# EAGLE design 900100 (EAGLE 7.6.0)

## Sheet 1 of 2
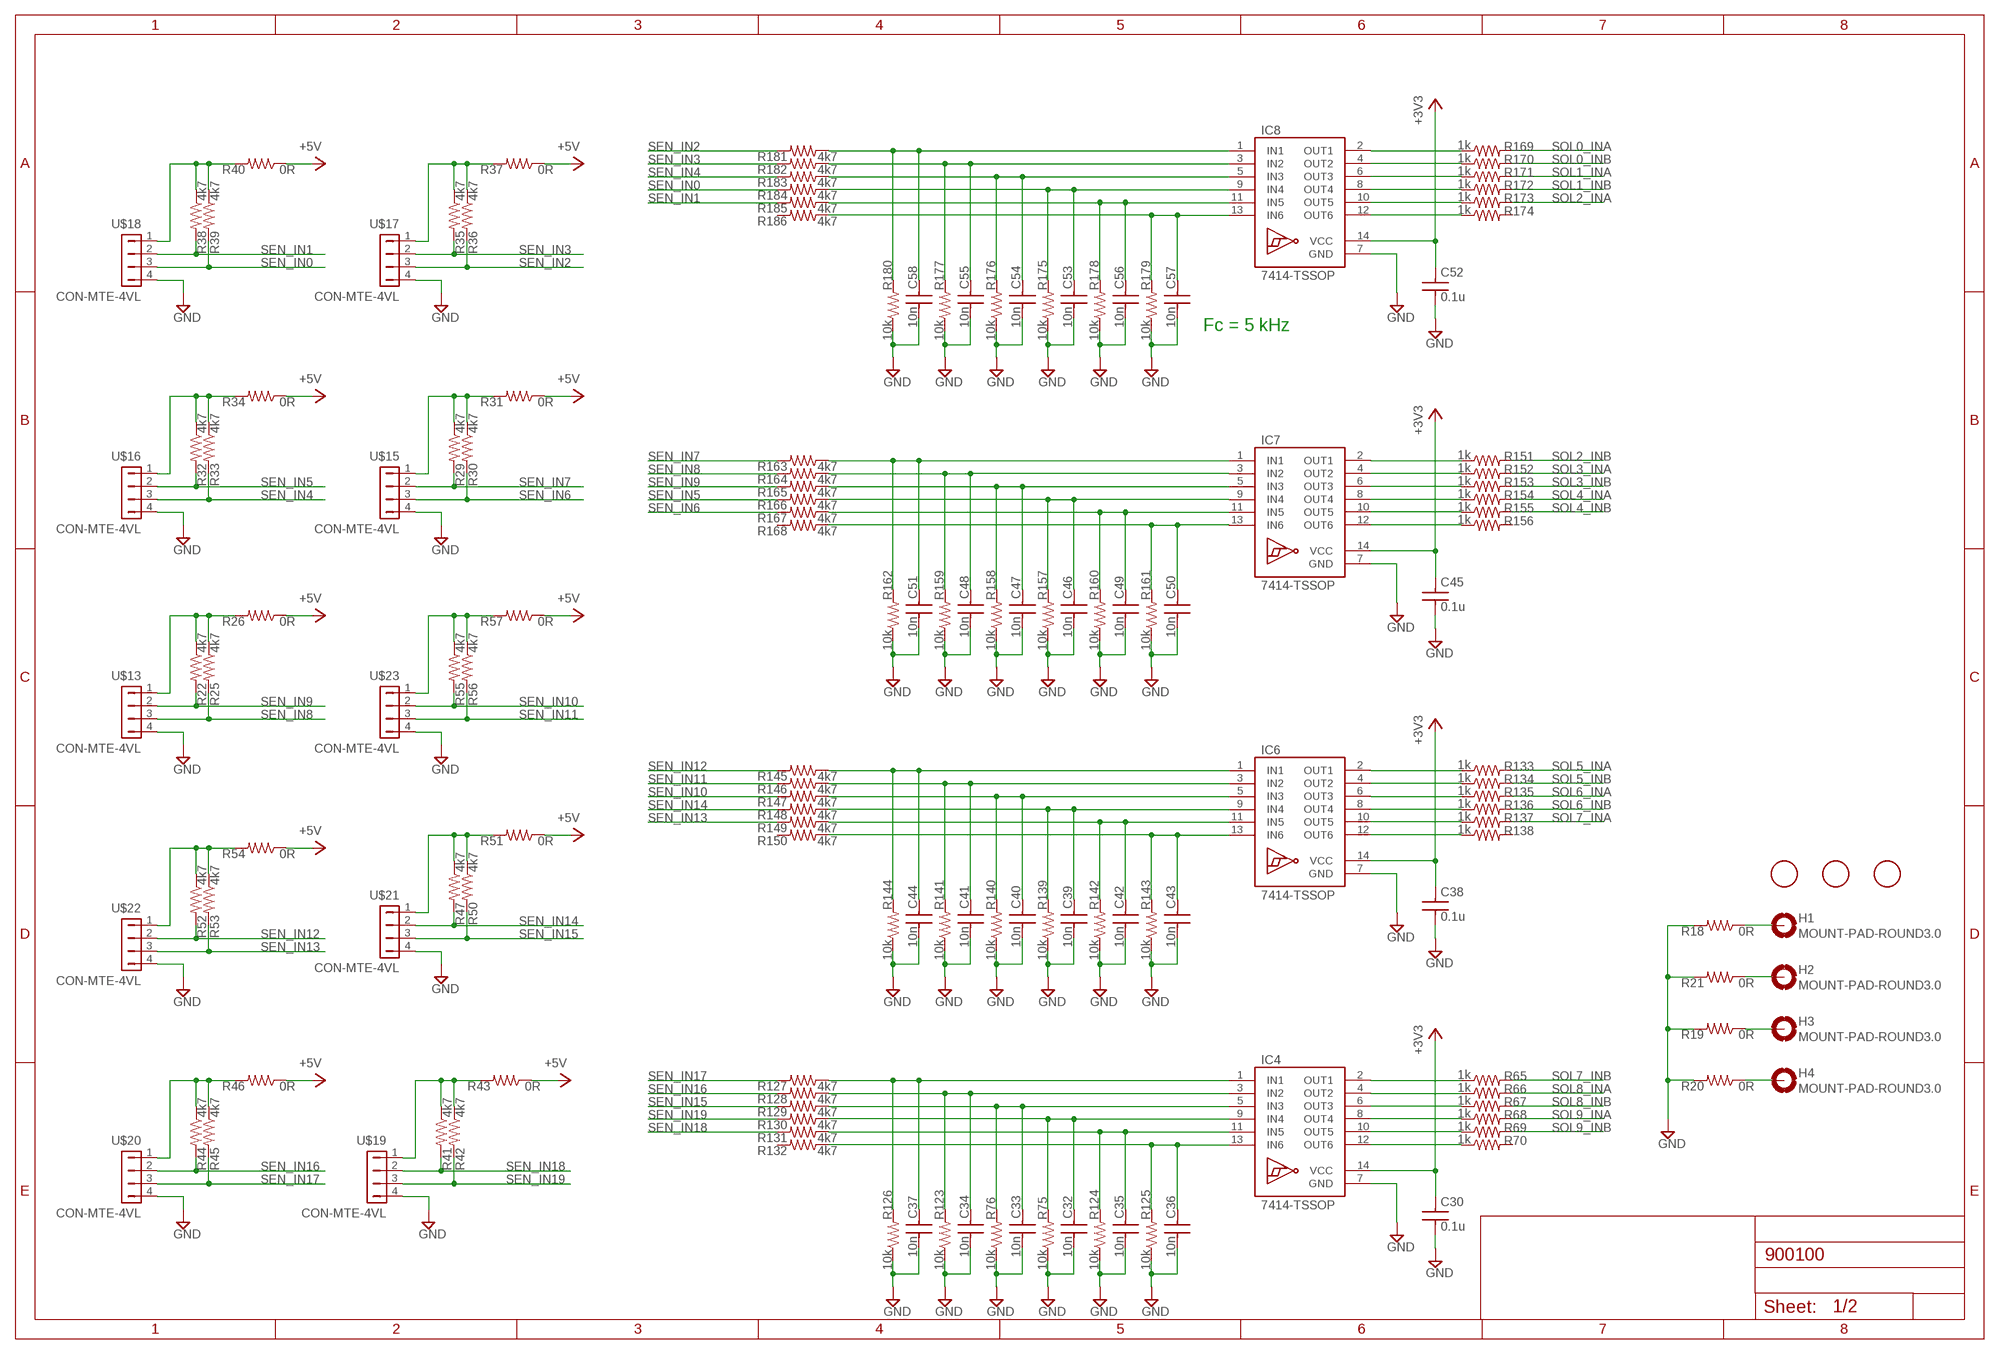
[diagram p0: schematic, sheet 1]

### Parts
C30  0.1u  C-USC0603K  [C0603K]
C32  10n  C-USC0603K  [C0603K]
C33  10n  C-USC0603K  [C0603K]
C34  10n  C-USC0603K  [C0603K]
C35  10n  C-USC0603K  [C0603K]
C36  10n  C-USC0603K  [C0603K]
C37  10n  C-USC0603K  [C0603K]
C38  0.1u  C-USC0603K  [C0603K]
C39  10n  C-USC0603K  [C0603K]
C40  10n  C-USC0603K  [C0603K]
C41  10n  C-USC0603K  [C0603K]
C42  10n  C-USC0603K  [C0603K]
C43  10n  C-USC0603K  [C0603K]
C44  10n  C-USC0603K  [C0603K]
C45  0.1u  C-USC0603K  [C0603K]
C46  10n  C-USC0603K  [C0603K]
C47  10n  C-USC0603K  [C0603K]
C48  10n  C-USC0603K  [C0603K]
C49  10n  C-USC0603K  [C0603K]
C50  10n  C-USC0603K  [C0603K]
C51  10n  C-USC0603K  [C0603K]
C52  0.1u  C-USC0603K  [C0603K]
C53  10n  C-USC0603K  [C0603K]
C54  10n  C-USC0603K  [C0603K]
C55  10n  C-USC0603K  [C0603K]
C56  10n  C-USC0603K  [C0603K]
C57  10n  C-USC0603K  [C0603K]
C58  10n  C-USC0603K  [C0603K]
H1  MOUNT-PAD-ROUND3.0  [3,0-PAD]
H2  MOUNT-PAD-ROUND3.0  [3,0-PAD]
H3  MOUNT-PAD-ROUND3.0  [3,0-PAD]
H4  MOUNT-PAD-ROUND3.0  [3,0-PAD]
IC4  7414-TSSOP  [TSSOP14-PW-4.40]
IC6  7414-TSSOP  [TSSOP14-PW-4.40]
IC7  7414-TSSOP  [TSSOP14-PW-4.40]
IC8  7414-TSSOP  [TSSOP14-PW-4.40]
R18  0R  R-US_R0603  [R0603]
R19  0R  R-US_R0603  [R0603]
R20  0R  R-US_R0603  [R0603]
R21  0R  R-US_R0603  [R0603]
R22  4k7  R-US_R0603  [R0603]
R25  4k7  R-US_R0603  [R0603]
R26  0R  R-US_R0603  [R0603]
R29  4k7  R-US_R0603  [R0603]
R30  4k7  R-US_R0603  [R0603]
R31  0R  R-US_R0603  [R0603]
R32  4k7  R-US_R0603  [R0603]
R33  4k7  R-US_R0603  [R0603]
R34  0R  R-US_R0603  [R0603]
R35  4k7  R-US_R0603  [R0603]
R36  4k7  R-US_R0603  [R0603]
R37  0R  R-US_R0603  [R0603]
R38  4k7  R-US_R0603  [R0603]
R39  4k7  R-US_R0603  [R0603]
R40  0R  R-US_R0603  [R0603]
R41  4k7  R-US_R0603  [R0603]
R42  4k7  R-US_R0603  [R0603]
R43  0R  R-US_R0603  [R0603]
R44  4k7  R-US_R0603  [R0603]
R45  4k7  R-US_R0603  [R0603]
R46  0R  R-US_R0603  [R0603]
R47  4k7  R-US_R0603  [R0603]
R50  4k7  R-US_R0603  [R0603]
R51  0R  R-US_R0603  [R0603]
R52  4k7  R-US_R0603  [R0603]
R53  4k7  R-US_R0603  [R0603]
R54  0R  R-US_R0603  [R0603]
R55  4k7  R-US_R0603  [R0603]
R56  4k7  R-US_R0603  [R0603]
R57  0R  R-US_R0603  [R0603]
R65  1k  R-US_R0603  [R0603]
R66  1k  R-US_R0603  [R0603]
R67  1k  R-US_R0603  [R0603]
R68  1k  R-US_R0603  [R0603]
R69  1k  R-US_R0603  [R0603]
R70  1k  R-US_R0603  [R0603]
R75  10k  R-US_R0603  [R0603]
R76  10k  R-US_R0603  [R0603]
R123  10k  R-US_R0603  [R0603]
R124  10k  R-US_R0603  [R0603]
R125  10k  R-US_R0603  [R0603]
R126  10k  R-US_R0603  [R0603]
R127  4k7  R-US_R0603  [R0603]
R128  4k7  R-US_R0603  [R0603]
R129  4k7  R-US_R0603  [R0603]
R130  4k7  R-US_R0603  [R0603]
R131  4k7  R-US_R0603  [R0603]
R132  4k7  R-US_R0603  [R0603]
R133  1k  R-US_R0603  [R0603]
R134  1k  R-US_R0603  [R0603]
R135  1k  R-US_R0603  [R0603]
R136  1k  R-US_R0603  [R0603]
R137  1k  R-US_R0603  [R0603]
R138  1k  R-US_R0603  [R0603]
R139  10k  R-US_R0603  [R0603]
R140  10k  R-US_R0603  [R0603]
R141  10k  R-US_R0603  [R0603]
R142  10k  R-US_R0603  [R0603]
R143  10k  R-US_R0603  [R0603]
R144  10k  R-US_R0603  [R0603]
R145  4k7  R-US_R0603  [R0603]
R146  4k7  R-US_R0603  [R0603]
R147  4k7  R-US_R0603  [R0603]
R148  4k7  R-US_R0603  [R0603]
R149  4k7  R-US_R0603  [R0603]
R150  4k7  R-US_R0603  [R0603]
R151  1k  R-US_R0603  [R0603]
R152  1k  R-US_R0603  [R0603]
R153  1k  R-US_R0603  [R0603]
R154  1k  R-US_R0603  [R0603]
R155  1k  R-US_R0603  [R0603]
R156  1k  R-US_R0603  [R0603]
R157  10k  R-US_R0603  [R0603]
R158  10k  R-US_R0603  [R0603]
R159  10k  R-US_R0603  [R0603]
R160  10k  R-US_R0603  [R0603]
R161  10k  R-US_R0603  [R0603]
R162  10k  R-US_R0603  [R0603]
R163  4k7  R-US_R0603  [R0603]
R164  4k7  R-US_R0603  [R0603]
R165  4k7  R-US_R0603  [R0603]
R166  4k7  R-US_R0603  [R0603]
R167  4k7  R-US_R0603  [R0603]
R168  4k7  R-US_R0603  [R0603]
R169  1k  R-US_R0603  [R0603]
R170  1k  R-US_R0603  [R0603]
R171  1k  R-US_R0603  [R0603]
R172  1k  R-US_R0603  [R0603]
R173  1k  R-US_R0603  [R0603]
R174  1k  R-US_R0603  [R0603]
R175  10k  R-US_R0603  [R0603]
R176  10k  R-US_R0603  [R0603]
R177  10k  R-US_R0603  [R0603]
R178  10k  R-US_R0603  [R0603]
R179  10k  R-US_R0603  [R0603]
R180  10k  R-US_R0603  [R0603]
R181  4k7  R-US_R0603  [R0603]
R182  4k7  R-US_R0603  [R0603]
R183  4k7  R-US_R0603  [R0603]
R184  4k7  R-US_R0603  [R0603]
R185  4k7  R-US_R0603  [R0603]
R186  4k7  R-US_R0603  [R0603]
U$7  FIDUCIAL  [FIDUCIAL_1MM]
U$13  CON-MTE-4VL  [MTE-100-4VL]
U$15  CON-MTE-4VL  [MTE-100-4VL]
U$16  CON-MTE-4VL  [MTE-100-4VL]
U$17  CON-MTE-4VL  [MTE-100-4VL]
U$18  CON-MTE-4VL  [MTE-100-4VL]
U$19  CON-MTE-4VL  [MTE-100-4VL]
U$20  CON-MTE-4VL  [MTE-100-4VL]
U$21  CON-MTE-4VL  [MTE-100-4VL]
U$22  CON-MTE-4VL  [MTE-100-4VL]
U$23  CON-MTE-4VL  [MTE-100-4VL]
U$60  FIDUCIAL  [FIDUCIAL_1MM]
U$62  FIDUCIAL  [FIDUCIAL_1MM]

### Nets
+3V3: C30.1 C38.1 C45.1 C52.1 IC4.14(VCC) IC6.14(VCC) IC7.14(VCC) IC8.14(VCC) ; also sheet 2
+5V: R26.1 R31.1 R34.1 R37.1 R40.1 R43.1 R46.1 R51.1 R54.1 R57.1 ; also sheet 2
GND [GND]: C30.2 C32.2 C33.2 C34.2 C35.2 C36.2 C37.2 C38.2 C39.2 C40.2 C41.2 C42.2 C43.2 C44.2 C45.2 C46.2 C47.2 C48.2 C49.2 C50.2 C51.2 C52.2 C53.2 C54.2 C55.2 C56.2 C57.2 C58.2 IC4.7(GND) IC6.7(GND) IC7.7(GND) IC8.7(GND) R18.2 R19.2 R20.2 R21.2 R75.1 R76.1 R123.1 R124.1 R125.1 R126.1 R139.1 R140.1 R141.1 R142.1 R143.1 R144.1 R157.1 R158.1 R159.1 R160.1 R161.1 R162.1 R175.1 R176.1 R177.1 R178.1 R179.1 R180.1 U$13.4 U$15.4 U$16.4 U$17.4 U$18.4 U$19.4 U$20.4 U$21.4 U$22.4 U$23.4 ; also sheet 2
N$1: IC4.4(OUT2) R66.1
N$2: IC4.2(OUT1) R65.1
N$3: IC6.6(OUT3) R135.1
N$5: IC6.4(OUT2) R134.1
N$6: IC6.2(OUT1) R133.1
N$7: IC7.2(OUT1) R151.1
N$8: IC7.4(OUT2) R152.1
N$9: IC8.2(OUT1) R169.1
N$10: IC8.4(OUT2) R170.1
N$16: R29.1 R30.1 R31.2 U$15.1
N$44: R22.1 R25.1 R26.2 U$13.1
N$58: H1.B3,0(MOUNT) R18.1
N$59: H3.B3,0(MOUNT) R19.1
N$60: H4.B3,0(MOUNT) R20.1
N$63: H2.B3,0(MOUNT) R21.1
N$64: R32.1 R33.1 R34.2 U$16.1
N$69: R35.1 R36.1 R37.2 U$17.1
N$70: R38.1 R39.1 R40.2 U$18.1
N$78: R41.1 R42.1 R43.2 U$19.1
N$79: R44.1 R45.1 R46.2 U$20.1
N$80: R47.1 R50.1 R51.2 U$21.1
N$81: R52.1 R53.1 R54.2 U$22.1
N$82: R55.1 R56.1 R57.2 U$23.1
N$106: IC4.12(OUT6) R70.1
N$107: IC4.10(OUT5) R69.1
N$108: IC4.8(OUT4) R68.1
N$109: IC4.6(OUT3) R67.1
N$110: C36.1 IC4.13(IN6) R125.2 R132.1
N$111: C35.1 IC4.11(IN5) R124.2 R131.1
N$112: C32.1 IC4.9(IN4) R75.2 R130.1
N$113: C33.1 IC4.5(IN3) R76.2 R129.1
N$115: C34.1 IC4.3(IN2) R123.2 R128.1
N$116: C37.1 IC4.1(IN1) R126.2 R127.1
N$163: IC6.12(OUT6) R138.1
N$164: IC6.10(OUT5) R137.1
N$165: IC6.8(OUT4) R136.1
N$167: C43.1 IC6.13(IN6) R143.2 R150.1
N$168: C42.1 IC6.11(IN5) R142.2 R149.1
N$169: C39.1 IC6.9(IN4) R139.2 R148.1
N$170: C40.1 IC6.5(IN3) R140.2 R147.1
N$171: C41.1 IC6.3(IN2) R141.2 R146.1
N$172: C44.1 IC6.1(IN1) R144.2 R145.1
N$179: IC7.12(OUT6) R156.1
N$180: IC7.10(OUT5) R155.1
N$181: IC7.8(OUT4) R154.1
N$182: IC7.6(OUT3) R153.1
N$183: C50.1 IC7.13(IN6) R161.2 R168.1
N$184: C49.1 IC7.11(IN5) R160.2 R167.1
N$185: C46.1 IC7.9(IN4) R157.2 R166.1
N$186: C47.1 IC7.5(IN3) R158.2 R165.1
N$187: C48.1 IC7.3(IN2) R159.2 R164.1
N$188: C51.1 IC7.1(IN1) R162.2 R163.1
N$195: IC8.12(OUT6) R174.1
N$196: IC8.10(OUT5) R173.1
N$197: IC8.8(OUT4) R172.1
N$198: IC8.6(OUT3) R171.1
N$199: C57.1 IC8.13(IN6) R179.2 R186.1
N$200: C56.1 IC8.11(IN5) R178.2 R185.1
N$201: C53.1 IC8.9(IN4) R175.2 R184.1
N$202: C54.1 IC8.5(IN3) R176.2 R183.1
N$203: C55.1 IC8.3(IN2) R177.2 R182.1
N$204: C58.1 IC8.1(IN1) R180.2 R181.1
SEN_IN0: R39.2 R184.2 U$18.3
SEN_IN1: R38.2 R185.2 U$18.2
SEN_IN2: R36.2 R181.2 U$17.3
SEN_IN3: R35.2 R182.2 U$17.2
SEN_IN4: R33.2 R183.2 U$16.3
SEN_IN5: R32.2 R166.2 U$16.2
SEN_IN6: R30.2 R167.2 U$15.3
SEN_IN7: R29.2 R163.2 U$15.2
SEN_IN8: R25.2 R164.2 U$13.3
SEN_IN9: R22.2 R165.2 U$13.2
SEN_IN10: R55.2 R147.2 U$23.2
SEN_IN11: R56.2 R146.2 U$23.3
SEN_IN12: R52.2 R145.2 U$22.2
SEN_IN13: R53.2 R149.2 U$22.3
SEN_IN14: R47.2 R148.2 U$21.2
SEN_IN15: R50.2 R129.2 U$21.3
SEN_IN16: R44.2 R128.2 U$20.2
SEN_IN17: R45.2 R127.2 U$20.3
SEN_IN18: R41.2 R131.2 U$19.2
SEN_IN19: R42.2 R130.2 U$19.3
SOL0_INA: R169.2 ; also sheet 2
SOL0_INB: R170.2 ; also sheet 2
SOL1_INA: R171.2 ; also sheet 2
SOL1_INB: R172.2 ; also sheet 2
SOL2_INA: R173.2 ; also sheet 2
SOL2_INB: R151.2 ; also sheet 2
SOL3_INA: R152.2 ; also sheet 2
SOL3_INB: R153.2 ; also sheet 2
SOL4_INA: R154.2 ; also sheet 2
SOL4_INB: R155.2 ; also sheet 2
SOL5_INA: R133.2 ; also sheet 2
SOL5_INB: R134.2 ; also sheet 2
SOL6_INA: R135.2 ; also sheet 2
SOL6_INB: R136.2 ; also sheet 2
SOL7_INA: R137.2 ; also sheet 2
SOL7_INB: R65.2 ; also sheet 2
SOL8_INA: R66.2 ; also sheet 2
SOL8_INB: R67.2 ; also sheet 2
SOL9_INA: R68.2 ; also sheet 2
SOL9_INB: R69.2 ; also sheet 2
Unconnected: R70.2 R132.2 R138.2 R150.2 R156.2 R168.2 R174.2 R186.2

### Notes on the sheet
- Fc = 5 kHz

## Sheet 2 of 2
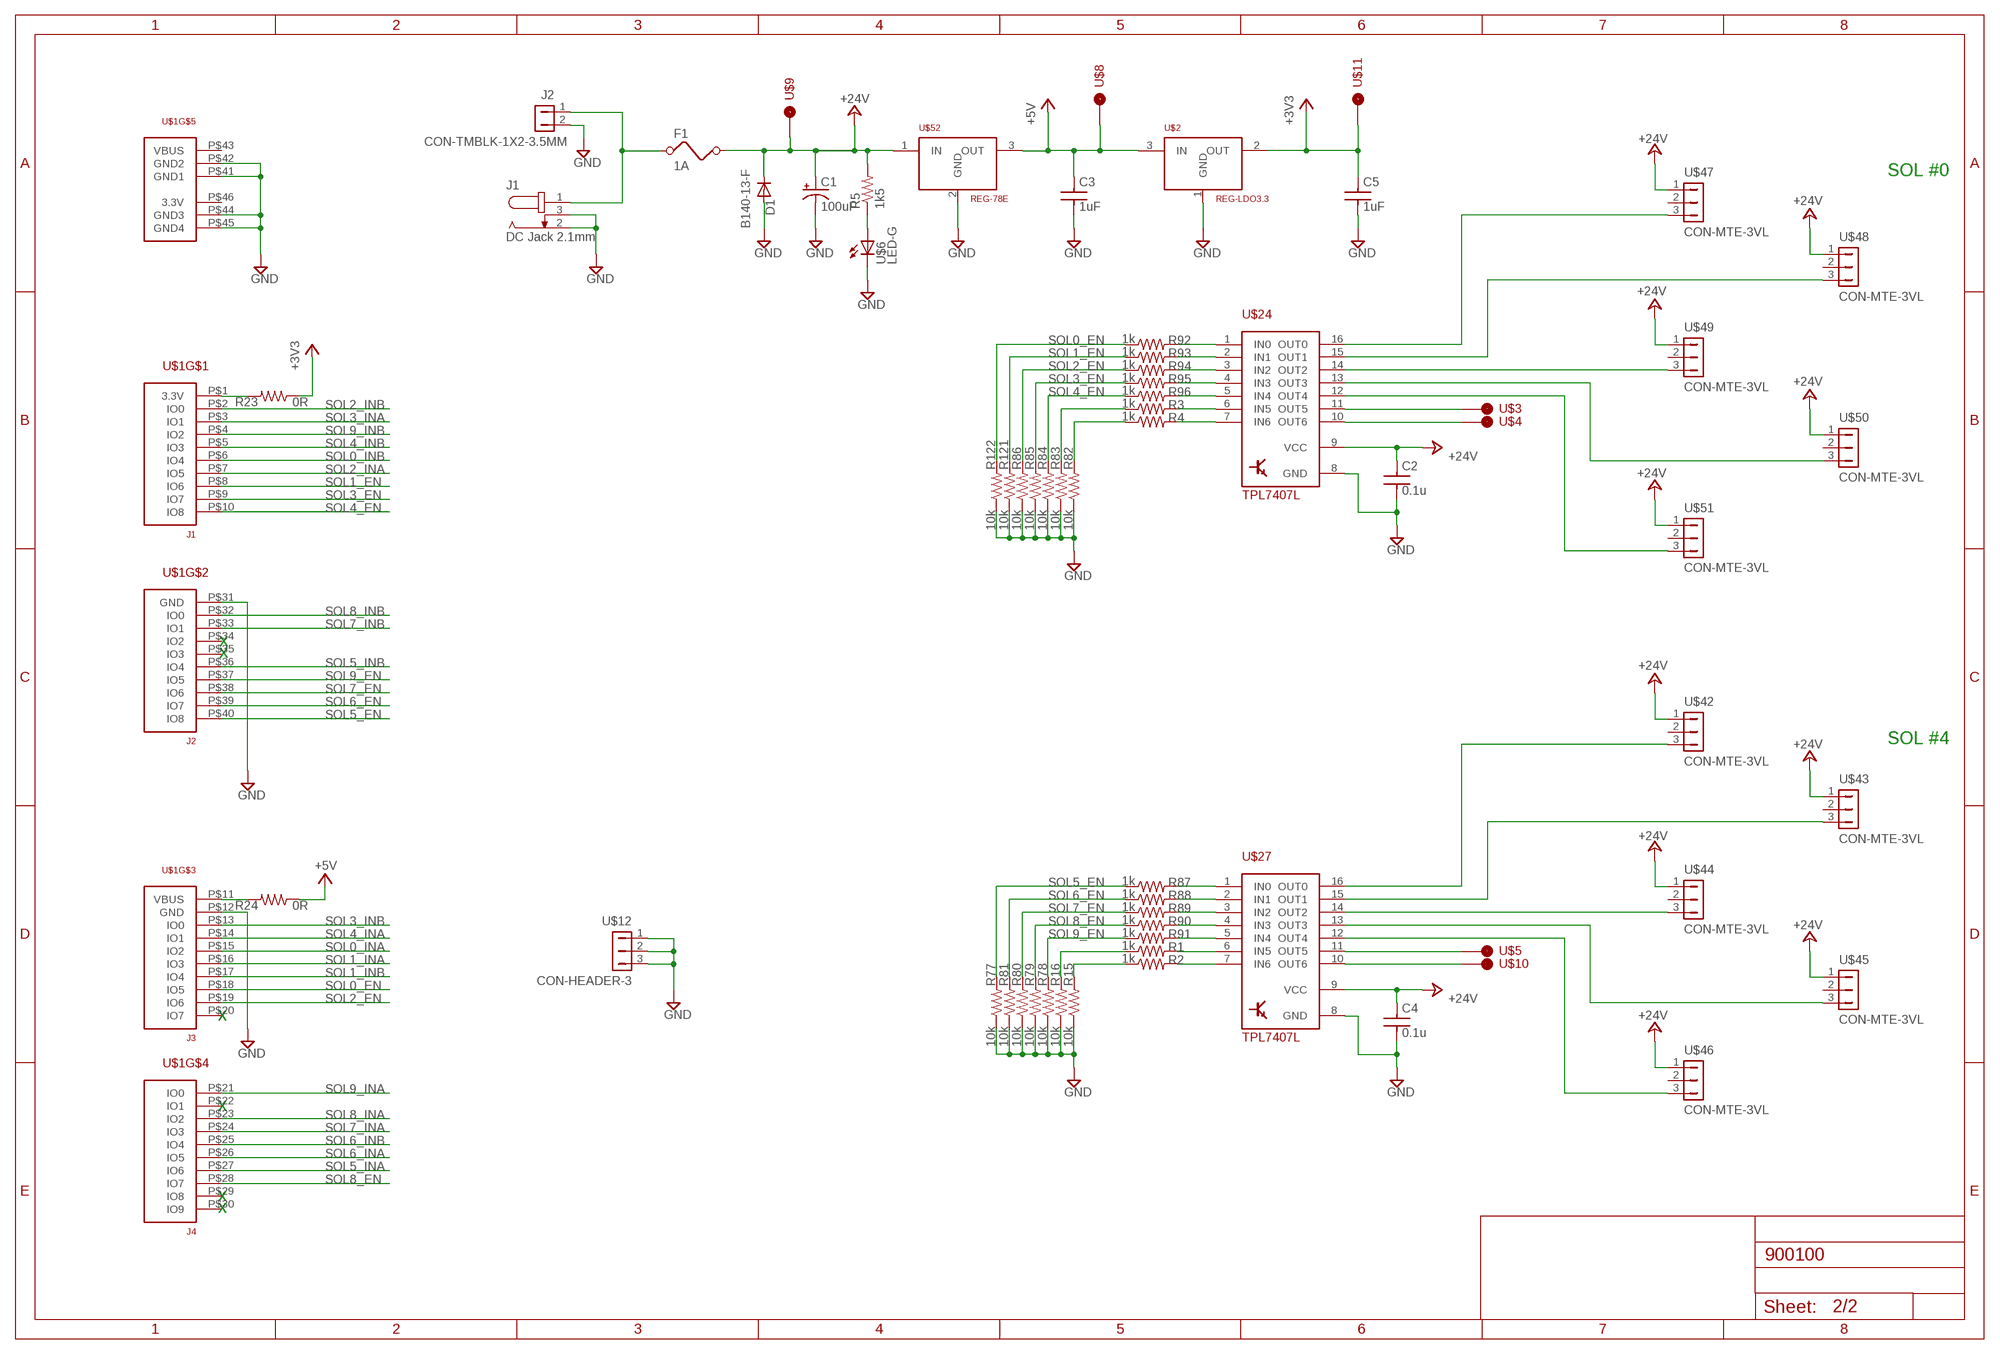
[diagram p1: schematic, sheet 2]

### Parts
C1  100uF  CPOL-USE5-10.5  [E5-10,5]
C2  0.1u  C-USC0603K  [C0603K]
C3  1uF  C-USC0603  [C0603]
C4  0.1u  C-USC0603K  [C0603K]
C5  1uF  C-USC0603  [C0603]
D1  B140-13-F  DIODE-DO214AC  [DO214AC]
F1  1A  FUSE  [FUSE_SMT]
J1  DC Jack 2.1mm  JACK-DC0  [SPC4077]
J2  CON-TMBLK-1X2-3.5MM  [1X2-3.5MM]
R1  1k  R-US_R0603  [R0603]
R2  1k  R-US_R0603  [R0603]
R3  1k  R-US_R0603  [R0603]
R4  1k  R-US_R0603  [R0603]
R5  1k5  R-USR1206  [R1206]
R15  10k  R-US_R0603  [R0603]
R16  10k  R-US_R0603  [R0603]
R23  0R  R-US_R0603  [R0603]
R24  0R  R-US_R0603  [R0603]
R77  10k  R-US_R0603  [R0603]
R78  10k  R-US_R0603  [R0603]
R79  10k  R-US_R0603  [R0603]
R80  10k  R-US_R0603  [R0603]
R81  10k  R-US_R0603  [R0603]
R82  10k  R-US_R0603  [R0603]
R83  10k  R-US_R0603  [R0603]
R84  10k  R-US_R0603  [R0603]
R85  10k  R-US_R0603  [R0603]
R86  10k  R-US_R0603  [R0603]
R87  1k  R-US_R0603  [R0603]
R88  1k  R-US_R0603  [R0603]
R89  1k  R-US_R0603  [R0603]
R90  1k  R-US_R0603  [R0603]
R91  1k  R-US_R0603  [R0603]
R92  1k  R-US_R0603  [R0603]
R93  1k  R-US_R0603  [R0603]
R94  1k  R-US_R0603  [R0603]
R95  1k  R-US_R0603  [R0603]
R96  1k  R-US_R0603  [R0603]
R121  10k  R-US_R0603  [R0603]
R122  10k  R-US_R0603  [R0603]
U$1  LAUNCHPAD-LM4F120  [LAUNCHPAD]
U$2  REG-LDO3.3  [SOT23]
U$3  TESTPOINT-TH  [TESTPOINT-TH]
U$4  TESTPOINT-TH  [TESTPOINT-TH]
U$5  TESTPOINT-TH  [TESTPOINT-TH]
U$6  LED-G  [R0603-POL]
U$8  TESTPOINT-TH  [TESTPOINT-TH]
U$9  TESTPOINT-TH  [TESTPOINT-TH]
U$10  TESTPOINT-TH  [TESTPOINT-TH]
U$11  TESTPOINT-TH  [TESTPOINT-TH]
U$12  CON-HEADER-3  [SIP-100-3V]
U$24  TPL7407L  [TSSOP16-PW-4.40]
U$27  TPL7407L  [TSSOP16-PW-4.40]
U$42  CON-MTE-3VL  [MTE-100-3VL]
U$43  CON-MTE-3VL  [MTE-100-3VL]
U$44  CON-MTE-3VL  [MTE-100-3VL]
U$45  CON-MTE-3VL  [MTE-100-3VL]
U$46  CON-MTE-3VL  [MTE-100-3VL]
U$47  CON-MTE-3VL  [MTE-100-3VL]
U$48  CON-MTE-3VL  [MTE-100-3VL]
U$49  CON-MTE-3VL  [MTE-100-3VL]
U$50  CON-MTE-3VL  [MTE-100-3VL]
U$51  CON-MTE-3VL  [MTE-100-3VL]
U$52  REG-78E  [SIP-100-3-78E]

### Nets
+3V3: C5.1 R23.1 U$2.2(OUT) U$11.P$1(TP) ; also sheet 1
+5V: C3.1 R24.1 U$2.3(IN) U$8.P$1(TP) U$52.3(OUT) ; also sheet 1
+24V: C1.+ C2.1 C4.1 D1.C F1.P$2 R5.2 U$9.P$1(TP) U$24.9(VCC) U$27.9(VCC) U$42.1 U$43.1 U$44.1 U$45.1 U$46.1 U$47.1 U$48.1 U$49.1 U$50.1 U$51.1 U$52.1(IN)
+24V_IN: F1.P$1 J1.1 J2.1
GND [GND]: C1.- C2.2 C3.2 C4.2 C5.2 D1.A J1.2 J1.3 J2.2 R15.1 R16.1 R77.1 R78.1 R79.1 R80.1 R81.1 R82.1 R83.1 R84.1 R85.1 R86.1 R121.1 R122.1 U$1.P$12(GND) U$1.P$31(GND) U$1.P$41(GND1) U$1.P$42(GND2) U$1.P$44(GND3) U$1.P$45(GND4) U$2.1(GND) U$6.2(C) U$12.1 U$12.2 U$12.3 U$24.8(GND) U$27.8(GND) U$52.2(GND) ; also sheet 1
N$4: R87.2 U$27.1(IN0)
N$11: R5.1 U$6.1(A)
N$13: U$24.14(OUT2) U$49.3
N$14: R92.2 U$24.1(IN0)
N$18: U$27.14(OUT2) U$44.3
N$19: R93.2 U$24.2(IN1)
N$20: R4.1 R82.2
N$21: R94.2 U$24.3(IN2)
N$22: R3.1 R83.2
N$23: U$3.P$1(TP) U$24.11(OUT5)
N$24: U$4.P$1(TP) U$24.10(OUT6)
N$25: U$27.16(OUT0) U$42.3
N$26: R2.1 R15.2
N$27: R1.1 R16.2
N$28: U$5.P$1(TP) U$27.11(OUT5)
N$29: U$10.P$1(TP) U$27.10(OUT6)
N$32: R3.2 U$24.6(IN5)
N$33: R4.2 U$24.7(IN6)
N$34: R2.2 U$27.7(IN6)
N$35: R1.2 U$27.6(IN5)
N$61: R95.2 U$24.4(IN3)
N$62: R23.2 U$1.P$1(3.3V)
N$65: R24.2 U$1.P$11(VBUS)
N$114: R96.2 U$24.5(IN4)
N$122: U$27.15(OUT1) U$43.3
N$124: U$27.13(OUT3) U$45.3
N$125: U$27.12(OUT4) U$46.3
N$126: U$24.16(OUT0) U$47.3
N$127: U$24.15(OUT1) U$48.3
N$129: U$24.13(OUT3) U$50.3
N$130: U$24.12(OUT4) U$51.3
N$131: R88.2 U$27.2(IN1)
N$132: R89.2 U$27.3(IN2)
N$133: R90.2 U$27.4(IN3)
N$134: R91.2 U$27.5(IN4)
SOL0_EN: R92.1 R122.2 U$1.P$18(IO5)
SOL0_INA: U$1.P$15(IO2) ; also sheet 1
SOL0_INB: U$1.P$6(IO4) ; also sheet 1
SOL1_EN: R93.1 R121.2 U$1.P$8(IO6)
SOL1_INA: U$1.P$16(IO3) ; also sheet 1
SOL1_INB: U$1.P$17(IO4) ; also sheet 1
SOL2_EN: R86.2 R94.1 U$1.P$19(IO6)
SOL2_INA: U$1.P$7(IO5) ; also sheet 1
SOL2_INB: U$1.P$2(IO0) ; also sheet 1
SOL3_EN: R85.2 R95.1 U$1.P$9(IO7)
SOL3_INA: U$1.P$3(IO1) ; also sheet 1
SOL3_INB: U$1.P$13(IO0) ; also sheet 1
SOL4_EN: R84.2 R96.1 U$1.P$10(IO8)
SOL4_INA: U$1.P$14(IO1) ; also sheet 1
SOL4_INB: U$1.P$5(IO3) ; also sheet 1
SOL5_EN: R77.2 R87.1 U$1.P$40(IO8)
SOL5_INA: U$1.P$27(IO6) ; also sheet 1
SOL5_INB: U$1.P$36(IO4) ; also sheet 1
SOL6_EN: R81.2 R88.1 U$1.P$39(IO7)
SOL6_INA: U$1.P$26(IO5) ; also sheet 1
SOL6_INB: U$1.P$25(IO4) ; also sheet 1
SOL7_EN: R80.2 R89.1 U$1.P$38(IO6)
SOL7_INA: U$1.P$24(IO3) ; also sheet 1
SOL7_INB: U$1.P$33(IO1) ; also sheet 1
SOL8_EN: R79.2 R90.1 U$1.P$28(IO7)
SOL8_INA: U$1.P$23(IO2) ; also sheet 1
SOL8_INB: U$1.P$32(IO0) ; also sheet 1
SOL9_EN: R78.2 R91.1 U$1.P$37(IO5)
SOL9_INA: U$1.P$21(IO0) ; also sheet 1
SOL9_INB: U$1.P$4(IO2) ; also sheet 1
Unconnected: U$1.P$20(IO7) U$1.P$22(IO1) U$1.P$29(IO8) U$1.P$30(IO9) U$1.P$34(IO2) U$1.P$35(IO3) U$1.P$43(VBUS) U$1.P$46(3.3V) U$42.2 U$43.2 U$44.2 U$45.2 U$46.2 U$47.2 U$48.2 U$49.2 U$50.2 U$51.2

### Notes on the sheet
- SOL #0
- x
- x
- SOL #4
- x
- x
- x
- x

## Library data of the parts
C1 = launchpad:CPOL-US: POLARIZED CAPACITOR, American symbol
C2-C5 C30 C32-C58 = launchpad:C-US: CAPACITOR, American symbol
D1 = launchpad:DIODE-: DIODE
F1 = launchpad:FUSE: FUSE
H1-H4 = launchpad:MOUNT-PAD-ROUND: MOUNTING PAD, round
IC4 IC6-IC8 = launchpad:7414-TSSOP: Hex schmitt trigger INVERTER
J1 = launchpad:JACK-DC: DC POWER JACK Power Jack, DC, Right Angle, Through Hole, Rated 5A at 16VDC, PC Terminals Distributor: Farnell (www.Farnell.de) Drawing: 84N1161.pdf / 84N1162.pdf Manufacturer: SPC Technology (www.spctechnology.com) Type: SPC4077 / SPC 4078; OC_FARNELL: unknown; OC_NEWARK: unknown
J2 = launchpad:CON-TMBLK-1X2: 3.5mm Terminal block
R1-R4 R65-R70 R87-R96 R133-R138 R151-R156 R169-R174 = launchpad:R-US_: RESISTOR, American symbol
R5 = launchpad:R-US: RESISTOR, American symbol
R15 R16 R18-R26 R29-R47 R50-R57 R75-R86 R121-R132 R139-R150 R157-R168 R175-R186 = rcl:R-US_: RESISTOR, American symbol
U$1 = launchpad:LAUNCHPAD-LM4F120
U$2 = launchpad:REG-LDO3.3
U$3-U$5 U$8-U$11 = launchpad:TESTPOINT-TH
U$6 = launchpad:LED-G
U$7 U$60 U$62 = launchpad:FIDUCIAL: For use by pick and place machines to calibrate the vision/machine, 1mm
U$12 = launchpad:CON-HEADER-3
U$13 U$15-U$23 = launchpad:CON-MTE-4VL
U$24 U$27 = launchpad:TPL7407L
U$42-U$51 = launchpad:CON-MTE-3VL
U$52 = launchpad:REG-78E

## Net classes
0 default: width 0.203 mm, drill 0.203 mm, clearance 0.203 mm
1 GND: width 0.203 mm, drill 0.305 mm, clearance 0.305 mm
2 +5V: width 0.305 mm, drill 0.305 mm, clearance 0.305 mm

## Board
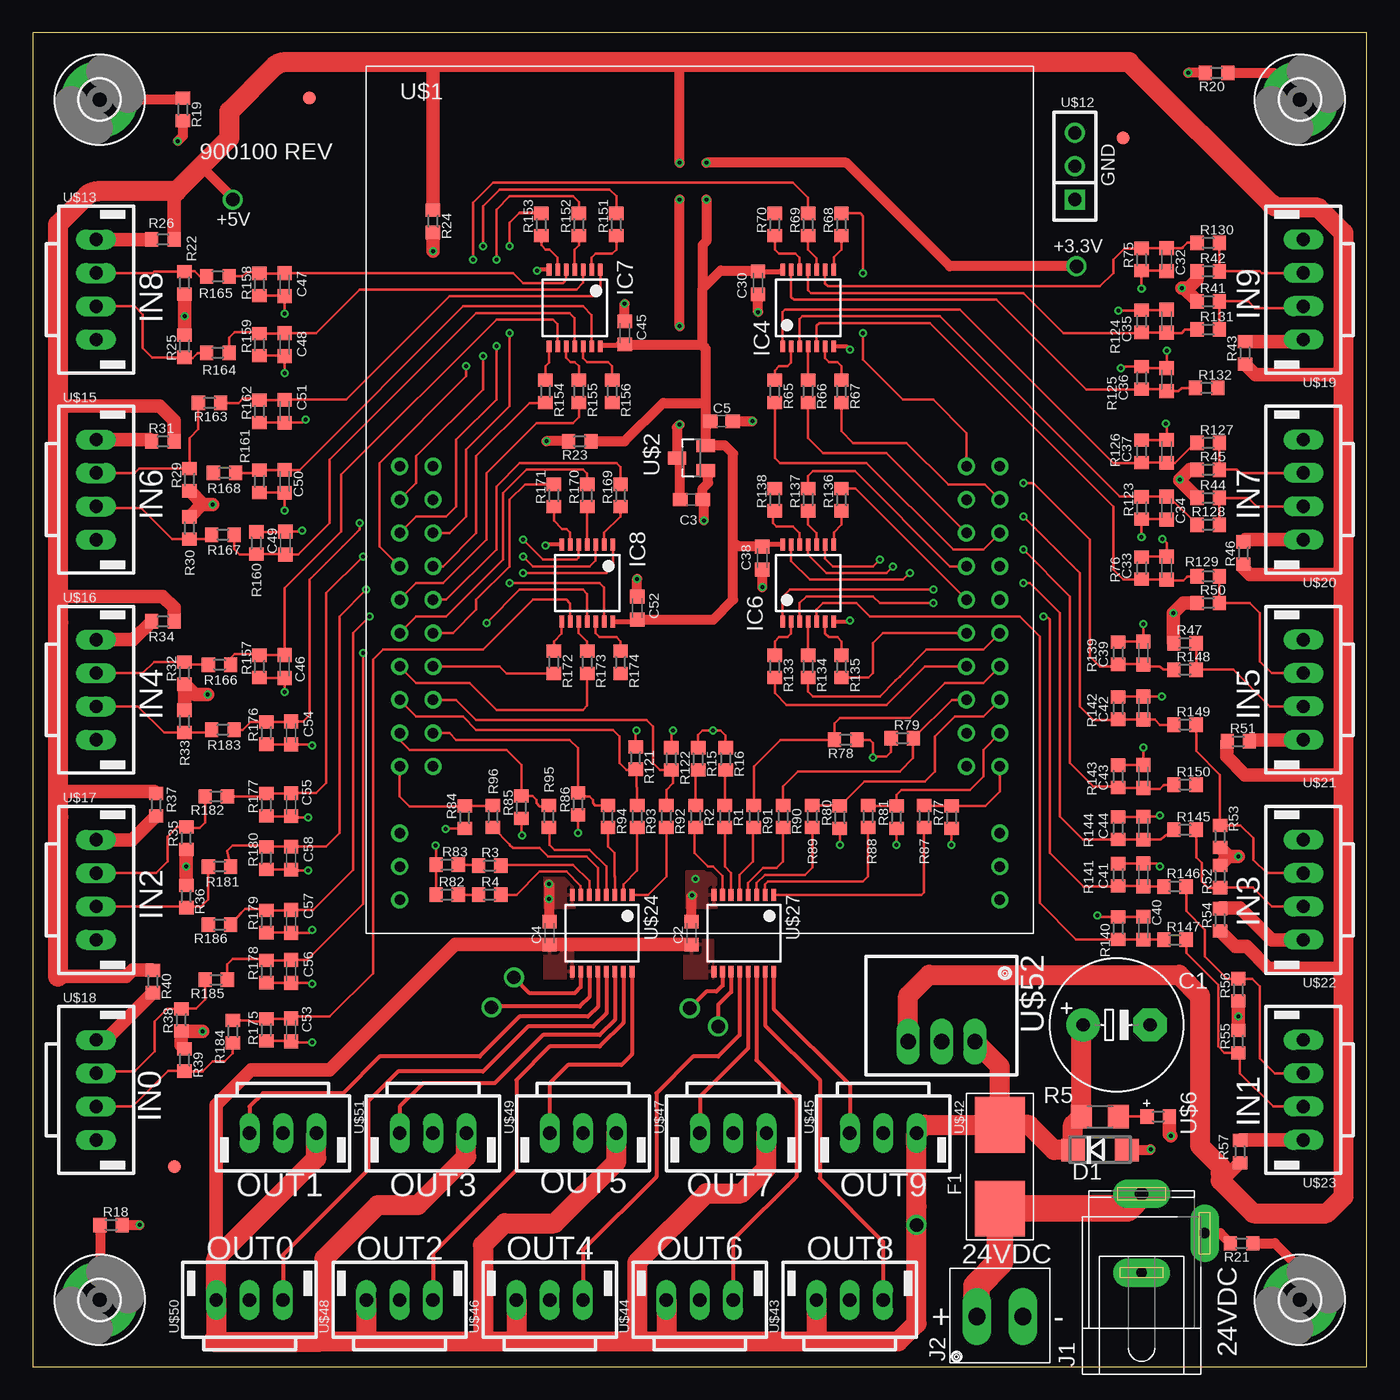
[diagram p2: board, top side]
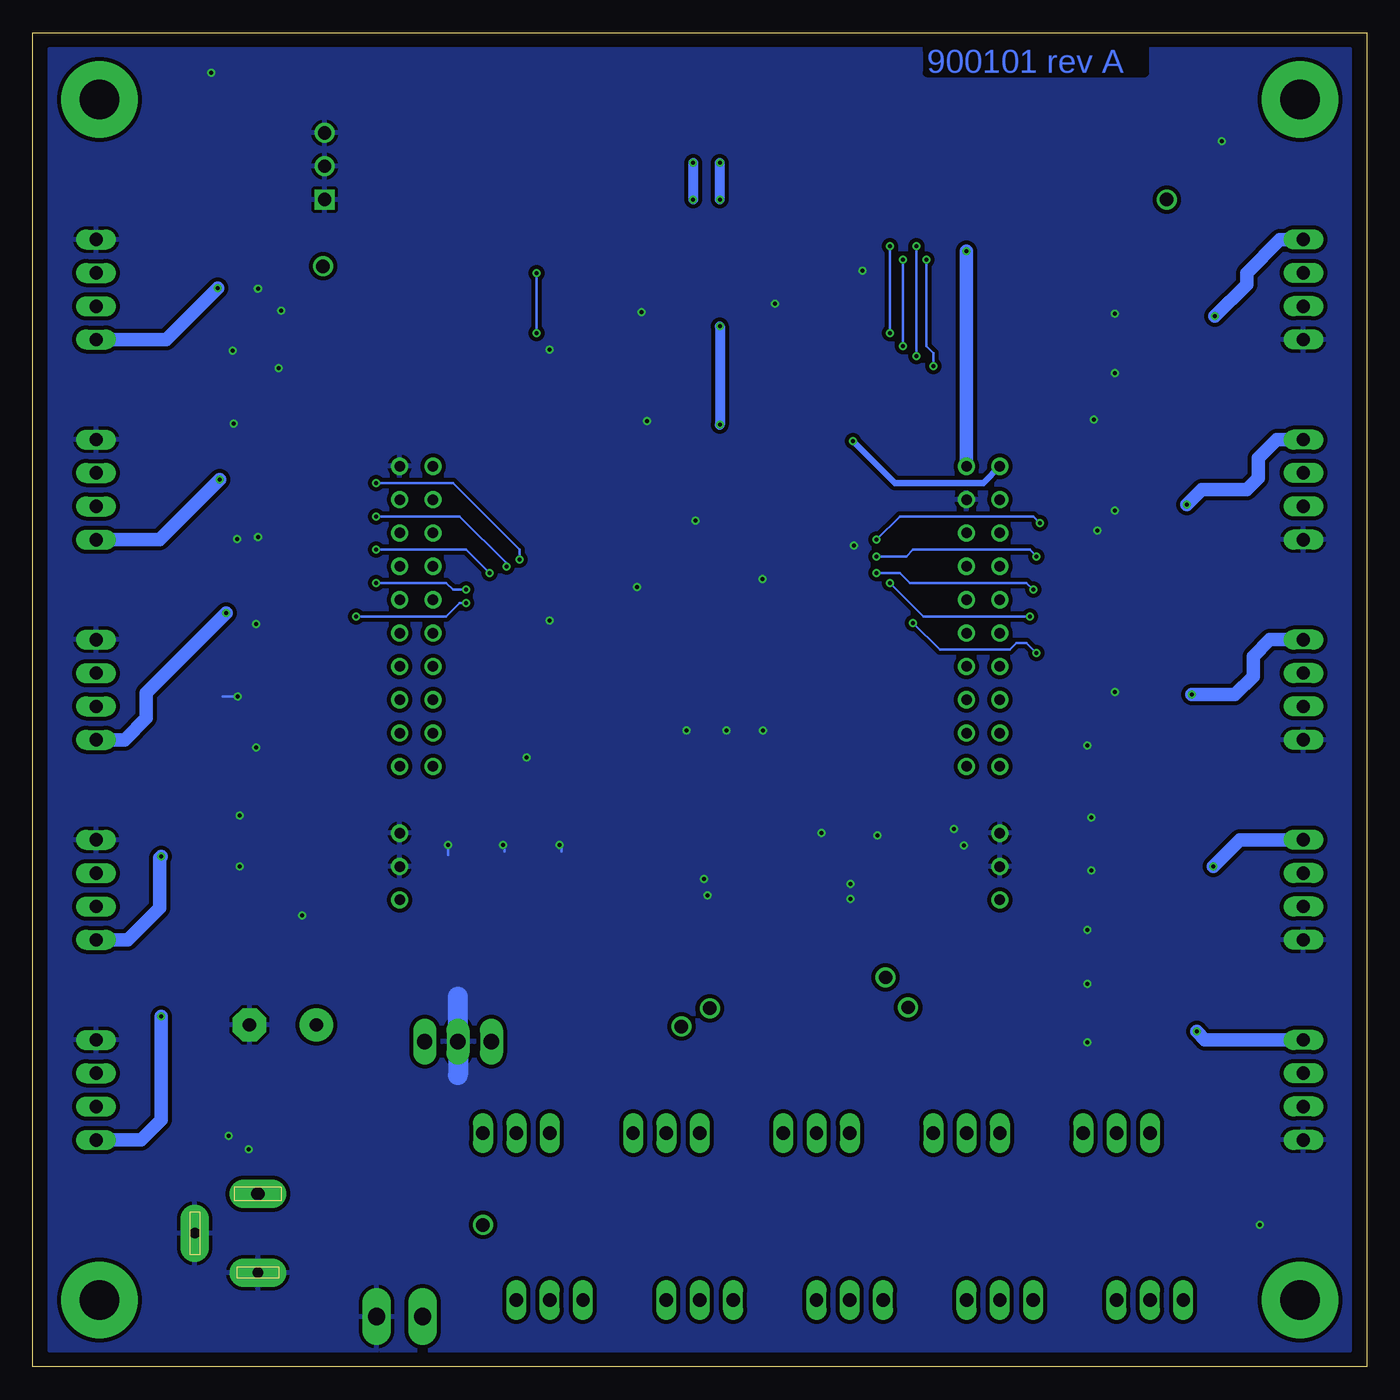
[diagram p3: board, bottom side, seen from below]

Size 101.6 x 101.6 mm. Coordinates in mm from the lower left corner, seen from the top.
Outline: 0,0 101.6,0 101.6,101.6 0,101.6 0,0
Copper layers (1*16): Top 0.035mm / dielectric 1.5mm / Bottom 0.035mm
Design rules "SeeedStudio_2layer_DRU_no_angle_20140221": minimum track width 6mil, minimum drill 12mil, track to track 6mil, track to pad 6mil, pad to pad 6mil, via to via 6mil, smd to smd 0mil, copper to edge 10mil, drill to drill 10mil, minimum pad ring 10mil, minimum via ring 6mil, stop-mask expansion 2mil, vias tented up to drill 100mil, thermal gap 10mil

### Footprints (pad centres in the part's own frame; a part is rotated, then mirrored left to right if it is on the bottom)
E5-10,5 = drill 1.016 pad 2.54: + -2.54,0 | drill 1.016 pad 2.54 octagon: - 2.54,0
C0603K = smd 1.05 x 1.08: 1 -0.875,0; 2 0.875,0
C0603 = smd 1.1 x 1: 1 -0.85,0; 2 0.85,0
DO214AC = smd 1.8 x 1.7: A 2.05,0; C -2.05,0
FUSE_SMT = smd 4.242 x 3.81: P$1 -3.188,0; P$2 3.188,0
3,0-PAD = drill 3 pad 5.842: B3,0 0,0
TSSOP14-PW-4.40 = smd 0.35 x 0.9: 1 -1.95,-2.925; 2 -1.3,-2.925; 3 -0.65,-2.925; 4 0,-2.925; 5 0.65,-2.925; 6 1.3,-2.925; 7 1.95,-2.925; 8 1.95,2.925; 9 1.3,2.925; 10 0.65,2.925; 11 0,2.925; 12 -0.65,2.925; 13 -1.3,2.925; 14 -1.95,2.925
SPC4077 = drill 1 pad 2.184 long: 1 3,0 | drill 0.8 pad 2.184 long: 2 -3,0; 3 0,-4.8
1X2-3.5MM = drill 1.321 pad 2.184 long: 1 1.75,0; 2 -1.75,0
R0603 = smd 1 x 1.1: 1 -0.85,0; 2 0.85,0
R1206 = smd 1.6 x 1.803: 1 -1.422,0; 2 1.422,0
LAUNCHPAD = drill 0.8: P$1 0,0; P$2 0,-2.54; P$3 0,-5.08; P$4 0,-7.62; P$5 0,-10.16; P$6 0,-12.7; P$7 0,-15.24; P$8 0,-17.78; P$9 0,-20.32; P$10 0,-22.86; P$11 2.54,0; P$12 2.54,-2.54; P$13 2.54,-5.08; P$14 2.54,-7.62; P$15 2.54,-10.16; P$16 2.54,-12.7; P$17 2.54,-15.24; P$18 2.54,-17.78; P$19 2.54,-20.32; P$20 2.54,-22.86; P$21 43.18,0; P$22 43.18,-2.54; P$23 43.18,-5.08; P$24 43.18,-7.62; P$25 43.18,-10.16; P$26 43.18,-12.7; P$27 43.18,-15.24; P$28 43.18,-17.78; P$29 43.18,-20.32; P$30 43.18,-22.86; P$31 45.72,0; P$32 45.72,-2.54; P$33 45.72,-5.08; P$34 45.72,-7.62; P$35 45.72,-10.16; P$36 45.72,-12.7; P$37 45.72,-15.24; P$38 45.72,-17.78; P$39 45.72,-20.32; P$40 45.72,-22.86; P$41 0,-27.94; P$42 0,-30.48; P$43 0,-33.02; P$44 45.72,-27.94; P$45 45.72,-30.48; P$46 45.72,-33.02
SOT23 = smd 1 x 1.4: 1 -0.95,-1.1; 2 0.95,-1.1; 3 0,1.1
TESTPOINT-TH = drill 1.016: P$1 0,0
R0603-POL = smd 1 x 1.1: 1 -0.85,0; 2 0.85,0
FIDUCIAL_1MM = smd 1 x 1: 1 0,0
SIP-100-3V = drill 1.016 square: 1 -2.54,0 | drill 1.016: 2 0,0; 3 2.54,0
MTE-100-4VL = drill 1.016 long: 1 -3.81,0; 2 -1.27,0; 3 1.27,0; 4 3.81,0
TSSOP16-PW-4.40 = smd 0.35 x 0.9: 1 -1.95,-2.925; 2 -1.3,-2.925; 3 -0.65,-2.925; 4 0,-2.925; 5 0.65,-2.925; 6 1.3,-2.925; 7 1.95,-2.925; 8 2.6,-2.925; 9 2.6,2.925; 10 1.95,2.925; 11 1.3,2.925; 12 0.65,2.925; 13 0,2.925; 14 -0.65,2.925; 15 -1.3,2.925; 16 -1.95,2.925
MTE-100-3VL = drill 1.016 long: 1 -2.54,0; 2 0,0; 3 2.54,0
SIP-100-3-78E = drill 1.168 long: 1 -2.54,0; 2 0,0; 3 2.54,0

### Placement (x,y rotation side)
C1  82.55,26.04 0 top
C2  50.16,33.02 90 top
C3  50.16,66.04 0 top
C4  39.37,33.02 90 top
C5  52.45,72.01 0 top
C30  55.24,82.55 270 top
C32  86.36,84.33 270 top
C33  86.36,60.83 90 top
C34  86.36,65.41 270 top
C35  86.36,79.63 90 top
C36  86.36,75.18 90 top
C37  86.36,69.72 90 top
C38  55.56,61.59 270 top
C39  84.58,54.36 90 top
C40  84.58,33.4 90 top
C41  84.58,37.47 90 top
C42  84.58,50.16 90 top
C43  84.58,44.96 90 top
C44  84.58,41.02 90 top
C45  45.09,78.74 90 top
C46  19.18,53.34 270 top
C47  19.18,82.42 270 top
C48  19.18,77.85 270 top
C49  19.24,62.74 90 top
C50  19.18,67.44 270 top
C51  19.18,72.77 270 top
C52  46.04,57.78 90 top
C53  19.68,25.65 270 top
C54  19.68,48.26 270 top
C55  19.68,42.8 270 top
C56  19.68,30.1 270 top
C57  19.68,33.91 270 top
C58  19.68,38.73 270 top
D1  81.28,16.51 0 top
F1  73.66,15.24 90 top
H1  5.08,5.08 0 top
H2  96.52,5.08 0 top
H3  5.08,96.52 0 top
H4  96.52,96.52 0 top
IC4  59.05,80.64 0 top
IC6  59.05,59.69 0 top
IC7  41.27,80.64 180 top
IC8  42.23,59.69 180 top
J1  84.45,10.16 90 top
J2  73.66,3.81 180 top
R1  52.7,41.91 270 top
R2  50.48,41.91 270 top
R3  34.8,38.16 0 top
R4  34.8,35.94 0 top
R5  81.28,19.05 180 top
R15  50.67,46.29 270 top
R16  52.77,46.29 270 top
R18  5.97,10.79 0 top
R19  11.43,95.76 270 top
R20  90.17,98.55 180 top
R21  92.08,9.4 180 top
R22  11.56,82.55 90 top
R23  41.66,70.48 180 top
R24  30.48,87.25 270 top
R25  11.56,77.72 270 top
R26  9.91,85.85 180 top
R29  11.94,67.56 90 top
R30  11.94,63.88 270 top
R31  9.91,70.48 180 top
R32  11.56,52.83 90 top
R33  11.56,49.15 270 top
R34  9.91,56.77 180 top
R35  11.68,40.26 90 top
R36  11.68,35.81 270 top
R37  9.4,42.8 270 top
R38  11.3,26.42 90 top
R39  11.56,23.37 270 top
R40  9.14,29.34 270 top
R41  89.53,81.15 0 top
R42  89.53,83.44 0 top
R43  92.33,77.22 90 top
R44  89.53,66.17 0 top
R45  89.53,68.33 0 top
R46  92.2,61.98 90 top
R47  87.76,55.12 0 top
R50  89.53,58.17 0 top
R51  91.82,47.62 0 top
R52  90.42,37.34 270 top
R53  90.42,40.39 90 top
R54  90.42,34.04 90 top
R55  91.82,24.77 270 top
R56  91.82,28.7 90 top
R57  91.95,16.38 90 top
R65  56.52,74.3 270 top
R66  59.05,74.3 270 top
R67  61.59,74.3 270 top
R68  61.59,87 90 top
R69  59.05,87 90 top
R70  56.52,87 90 top
R75  84.45,84.33 90 top
R76  84.45,60.83 270 top
R77  69.98,41.85 90 top
R78  61.91,47.75 180 top
R79  66.23,47.88 0 top
R80  61.47,41.85 90 top
R81  65.79,41.85 90 top
R82  31.56,35.94 0 top
R83  31.56,38.23 0 top
R84  32.89,41.85 90 top
R85  37.21,42.61 90 top
R86  41.53,42.86 90 top
R87  67.88,41.91 270 top
R88  63.63,41.91 270 top
R89  59.37,41.91 270 top
R90  57.15,41.91 270 top
R91  54.93,41.91 270 top
R92  48.26,41.91 270 top
R93  46.04,41.91 270 top
R94  43.81,41.91 270 top
R95  39.31,41.91 270 top
R96  35.05,41.91 270 top
R121  45.91,46.35 270 top
R122  48.64,46.29 270 top
R123  84.45,65.41 90 top
R124  84.45,79.63 270 top
R125  84.45,75.31 270 top
R126  84.45,69.72 270 top
R127  89.53,70.36 0 top
R128  89.53,64.14 0 top
R129  89.53,60.2 0 top
R130  89.53,85.6 0 top
R131  89.53,78.99 0 top
R132  89.41,74.55 0 top
R133  56.52,53.34 270 top
R134  59.05,53.34 270 top
R135  61.59,53.34 270 top
R136  61.59,66.04 90 top
R137  59.05,66.04 90 top
R138  56.52,66.04 90 top
R139  82.68,54.36 270 top
R140  82.68,33.4 270 top
R141  82.68,37.47 270 top
R142  82.68,50.16 270 top
R143  82.68,44.96 270 top
R144  82.68,41.02 270 top
R145  87.76,40.89 0 top
R146  87,36.58 0 top
R147  87,32.51 0 top
R148  87.76,53.09 0 top
R149  87.76,48.9 0 top
R150  87.76,44.32 0 top
R151  44.45,87 90 top
R152  41.59,87 90 top
R153  38.73,87 90 top
R154  39.05,74.3 270 top
R155  41.59,74.3 270 top
R156  44.13,74.3 270 top
R157  17.27,53.34 90 top
R158  17.27,82.42 90 top
R159  17.27,77.85 90 top
R160  17.02,62.74 270 top
R161  17.27,67.44 90 top
R162  17.27,72.77 90 top
R163  13.46,73.41 180 top
R164  14.1,77.22 180 top
R165  14.1,83.06 180 top
R166  14.22,53.47 180 top
R167  14.48,63.37 180 top
R168  14.61,68.07 180 top
R169  44.77,66.36 90 top
R170  42.23,66.36 90 top
R171  39.69,66.36 90 top
R172  39.69,53.66 270 top
R173  42.23,53.66 270 top
R174  44.77,53.66 270 top
R175  17.78,25.65 90 top
R176  17.78,48.26 90 top
R177  17.78,42.8 90 top
R178  17.78,30.1 90 top
R179  17.78,33.91 90 top
R180  17.78,38.73 90 top
R181  14.22,38.1 180 top
R182  13.97,43.43 180 top
R183  14.48,48.51 180 top
R184  15.24,25.53 270 top
R185  13.97,29.46 180 top
R186  14.22,33.66 180 top
U$1  27.94,68.58 0 top
U$2  50.16,69.22 90 top
U$3  34.92,27.37 0 top
U$4  36.64,29.65 0 top
U$5  52.2,25.91 0 top
U$6  85.72,19.05 0 top
U$7  83.06,93.6 0 top
U$8  15.24,88.9 0 top
U$9  67.31,10.79 0 top
U$10  50.04,27.3 0 top
U$11  79.5,83.82 0 top
U$12  79.38,91.44 90 top
U$13  4.83,82.04 270 top
U$15  4.83,66.8 270 top
U$16  4.83,51.56 270 top
U$17  4.83,36.32 270 top
U$18  4.83,21.08 270 top
U$19  96.77,82.04 90 top
U$20  96.77,66.8 90 top
U$21  96.77,51.56 90 top
U$22  96.77,36.32 90 top
U$23  96.77,21.08 90 top
U$24  43.69,33.02 180 top
U$27  54.48,33.02 180 top
U$42  64.77,17.78 180 top
U$43  62.23,5.08 0 top
U$44  50.8,5.08 0 top
U$45  53.34,17.78 180 top
U$46  39.37,5.08 0 top
U$47  41.91,17.78 180 top
U$48  27.94,5.08 0 top
U$49  30.48,17.78 180 top
U$50  16.51,5.08 0 top
U$51  19.05,17.78 180 top
U$52  69.22,24.77 180 top
U$60  21.08,96.65 0 top
U$62  10.79,15.24 0 top

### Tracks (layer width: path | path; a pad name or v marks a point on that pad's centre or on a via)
+3V3  (via drill 0.3)
  Top 0.203: 51.39,72.01 C5.1
  Top 0.381: C30.1 56.96,83.42 IC4.14 | C45.1 44.53,77.86 44.45,77.79 43.29,77.79 IC7.14 | IC6.14 55.71,62.62 C38.1 | IC8.14 45.89,56.77 C52.1
  Top 0.762: C38.1 53.73,62.47 53.34,62.87 | 53.34,62.87 53.34,69.53 52.7,70.17 U$2.2 51.27,71.88 | C52.1 51.83,56.91 53.34,58.42 53.34,62.87 | 51.02,77.79 51.02,82.13 | 51.02,82.13 52.39,83.5 55.17,83.5 C30.1 | C45.1 50.94,77.86 51.02,77.79 | 51.27,71.88 51.27,73.41 | 51.27,73.41 51.27,77.54 51.02,77.79 | 51.39,72.01 51.27,71.88 | R23.1 45.09,70.48 48.01,73.41 51.27,73.41 | U$11.P$1 69.85,83.82 61.98,91.69 v51.31,91.69 | v51.31,88.9 51.31,85.72 51.02,85.43 51.02,82.13
  Bottom 0.762: v51.31,91.69 v51.31,88.9
+5V  (via drill 0.3)
  Top 0.762: C3.1 49.31,68.97 U$2.3 49.06,71.54 v49.28,71.75 | v49.28,79.25 v49.28,88.9 | v49.28,91.69 49.28,99.38 | U$8.P$1 15.24,89.03 12.83,91.44
  Top 1.016: 2.2,41.87 1.91,42.16 | 2.2,56.68 1.91,56.39 | 1.91,73.66 2.41,73.15 9.65,73.15 10.76,72.05 R31.1 | 4.97,89.53 4.97,89.35 | R24.1 30.48,99.38 | 10.92,89.53 10.76,89.37 R26.1 | 1.91,58.93 2.16,58.67 9.91,58.67 10.76,57.82 R34.1 | R40.1 9.11,30.23 7.62,30.23 7.11,29.72 1.91,29.72 | R57.1 91.15,14.73 90.49,14.73 | R54.1 91.61,32 92.46,32 94.11,30.35 99.82,30.35 | R51.1 90.93,47.59 90.93,46.48 92.33,45.09 99.82,45.09 | R46.1 92.2,60.83 92.71,60.33 99.69,60.33 99.82,60.45 | R43.1 93.13,75.56 99.82,75.56 | R37.1 9.23,43.81 1.91,43.81
  Top 1.524: U$52.3 66.67,28.26 68.26,29.84 87.31,29.84 88.9,28.26 88.9,16.83 90.49,15.24 90.49,14.73 90.49,14.16 92.96,11.68 98.55,11.68 99.82,12.95 99.82,30.35 99.82,45.09 99.82,60.45 99.82,75.56 99.82,86.36 97.92,88.27 95.14,88.27 arc-45 94.24,88.64 83.5,99.38 49.28,99.38 30.48,99.38 19.26,99.38 arc45 18.36,99.01 14.99,95.63 14.99,93.6 12.83,91.44 10.92,89.53 4.97,89.53 arc45 4.07,89.16 1.91,87 1.91,73.66 1.91,58.93 1.91,56.39 1.91,43.81 1.91,42.16 1.91,29.72
  Bottom 0.762: v49.28,88.9 v49.28,91.69 | v49.28,79.25 v49.28,71.75
+24V
  Top 1.016: C2.1 C4.1 32.15,32.15 22.61,22.61 16.64,22.61 13.97,19.94 13.97,8.26 14.61,8.89 14.86,8.89
  Top 1.524: F1.P$2 73.67,18.41 75.88,18.41 77.79,16.51 D1.C 79.23,18.42 R5.2 79.86,25.88 C1.+ | F1.P$2 73.66,22.86 U$52.1 | 59.69,1.91 65.91,1.91 67.31,3.3 U$9.P$1 67.31,12.19 U$42.1 67.96,18.43 F1.P$2 | 59.69,1.91 48.13,1.91 | 48.13,1.91 46.04,1.91 | 46.04,1.91 36.83,1.91 | 36.83,1.91 34.61,1.91 | 34.61,1.91 25.65,1.91 | 25.65,1.91 21.91,1.91 | 21.91,1.91 13.72,1.91 13.97,2.16 U$50.1 13.97,8.26 21.59,15.88 U$51.1 | 21.91,1.91 22.23,2.22 22.23,8.26 26.29,12.32 29.34,12.32 33.02,16 U$49.1 | 34.61,1.91 34.29,2.22 34.29,9.27 35.94,10.92 39.75,10.92 44.45,15.62 U$47.1 | 46.04,1.91 46.04,7.94 51.31,13.21 53.98,13.21 55.88,15.11 U$45.1 | U$48.1 25.4,2.16 25.65,1.91 | U$46.1 36.83,1.91 | U$44.1 48.26,2.03 48.13,1.91 | U$43.1 59.69,1.91
  pour Top: 49.66,32.51 49.66,29.59 51.82,29.59 51.82,32.51 49.78,32.51
  pour Top: 38.99,32.51 38.99,29.59 41.15,29.59 41.15,32.51 39.12,32.51
+24V_IN
  Top 2.032: J2.1 71.86,6.14 73.66,7.94 F1.P$1 73.67,12.06 77.47,12.06 78.11,12.06 83.36,12.06 J1.1
GND  (via drill 0.3)
  Top 0.203: v86.36,77.41 C36.2 84.56,76.06 R125.1 82.96,76.16 v82.87,76.07 | v84.45,82.11 R75.1 86.33,83.48 C32.2 | v86.04,63.06 86.36,62.74 C33.2 84.48,61.71 R76.1 | v84.45,63.18 R123.1 86.33,64.56 C34.2 | v84.58,56.58 C39.2 82.7,55.23 R139.1 | R143.1 82.7,45.83 C43.2 v84.58,47.18 | R126.1 86.33,70.57 C37.2 86.36,71.75 v86.3,71.82 | v81.09,34.35 81.19,34.25 R140.1 84.56,34.25 C40.2 | v85.85,38.1 85.61,38.34 C41.2 84.56,38.31 R141.1 | R144.1 84.56,41.87 C44.2 85.78,41.9 v85.85,41.97 | R179.1 19.66,33.06 C57.2 21.03,33.03 v21.27,33.27 | R162.1 19.15,71.92 C51.2 20.52,71.9 v20.77,72.14 | R178.1 17.8,29.22 C56.2 21.2,29.22 v21.27,29.15 | R158.1 19.15,81.57 C47.2 v19.18,80.2 | R161.1 19.15,66.59 C50.2 v19.18,65.22 | v20.51,63.69 20.43,63.61 C49.2 19.21,63.59 R160.1 | 19.25,52.39 C46.2 | C46.2 17.3,52.47 R157.1 | R175.1 19.66,24.8 C53.2 19.76,24.7 v21.27,24.7 | R180.1 19.66,37.88 C58.2 19.76,37.78 v20.95,37.78 | v20.95,41.85 19.76,41.85 C55.2 17.8,41.92 R177.1 | R176.1 19.66,47.41 C54.2 21.2,47.38 v21.27,47.31 | v19.18,51.37 C46.2 | R79.1 65.38,46.84 65.02,46.48 64.07,46.48 v64.01,46.42 64.01,47.5 63.75,47.75 R78.1 | R15.1 50.67,48.13 50.99,48.45 v51.82,48.45 52.39,48.45 52.77,48.07 R16.1 | R122.1 48.64,48.32 v48.77,48.45 | R121.1 45.91,48.39 v45.97,48.45 | R85.1 37.21,40.51 v37.27,40.45 | R82.1 R83.1 30.71,39.65 v30.67,39.69 | R84.1 31.47,41 v31.43,40.96 | C35.2 86.33,80.48 R124.1 84.43,80.45 v82.68,80.45 | R86.1 v41.53,40.64 | R77.1 v69.98,39.75 | R80.1 v61.47,39.75 | R81.1 v65.79,39.75 | R142.1 82.7,51.04 C42.2 84.6,51.05 v85.98,51.05 | R159.1 19.15,77 C48.2 v19.18,75.69
  Top 0.305: IC6.7 62.16,56.77 | IC8.7 39.12,62.62 | IC4.7 61.98,77.72 v62.23,77.47 | IC7.7 38.48,83.57 v38.42,83.5
  Top 0.381: 62.16,56.77 v62.23,56.83 | 39.12,62.62 v39.05,62.55
  Top 0.762: v55.56,59.37 C38.2 | C52.2 v46.04,60.01 | v51.12,64.45 51.12,65.94 C3.2 51.02,66.89 51.44,67.31 51.44,68.09 U$2.1 | C45.2 v45.09,80.96 | v55.24,80.33 C30.2 | C2.2 50.16,35.81 v50.23,35.88 | v39.31,36.77 v39.31,35.62 39.31,33.96 C4.2 | D1.A 85.09,16.51 v85.15,16.57 | C5.2 v54.8,72.01 | R19.2 11.43,93.73 v11.05,93.34 | R20.2 v88.01,98.55 | R18.2 v8.13,10.79 | R21.2 90.46,10.16 J1.3
  Top 1.016: U$6.2 86.58,17.69 v86.68,17.59
  Bottom 0.203: v69.98,39.75 69.98,38.99 | v61.47,39.75 61.34,39.88 61.34,39.24 | v65.79,39.75 65.66,39.88 65.66,39.24 | v85.98,51.05 87.12,51.05 | v19.18,75.69 19.3,75.82
  Bottom 1.524: 69.22,28.19 U$52.2 69.22,22.23
  other vias: 50.48,37.15
  pour Bottom: 1.27,100.33 100.33,100.33 100.33,1.27 1.27,1.27
  pour Top: 38.99,37.59 41.27,37.59 41.27,34.92 38.99,34.92
  pour Top: 49.78,37.72 52.07,37.72 52.07,34.92 49.78,34.92
N$1
  Top 0.203: IC4.4 R66.1
N$2
  Top 0.203: IC4.2 57.76,76.49 57.47,76.2 56.83,76.2 56.52,75.88 R65.1
N$3
  Top 0.203: IC6.6 60.35,55.85 60.64,55.56 61.28,55.56 61.59,55.24 R135.1
N$4
  Top 0.203: 67.94,41 R87.2 67.88,36.13 67.69,35.94 67.69,35.95 U$27.1
N$5
  Top 0.203: IC6.4 R134.1
N$6
  Top 0.203: IC6.2 57.76,55.85 57.47,55.56 56.83,55.56 56.52,55.24 R133.1
N$7
  Top 0.203: IC7.2 42.58,84.48 42.86,84.77 44.13,84.77 44.45,85.09 R151.1
N$8
  Top 0.203: IC7.4 41.27,85.09 41.59,85.41 R152.1
N$9
  Top 0.203: IC8.2 43.53,63.53 44.77,64.77 R169.1
N$10
  Top 0.203: R170.1 IC8.4
N$11
  Top 0.203: U$6.1 R5.1
N$13
  Top 0.305: U$24.14 44.34,26.43 43.18,25.27 38.86,25.27 35.18,21.59 29.72,21.59 27.94,19.81 U$49.3
N$14
  Top 0.203: U$24.1 46.87,35.95 48.26,37.34 R92.2
N$16  (via drill 0.3)
  Top 1.016: R31.2 8.93,70.61 U$15.1 | R30.1 12.87,65.66 v13.72,65.66 12.99,65.66 R29.1
  Bottom 1.016: v13.72,65.66 12.57,66.8 9.14,66.8 8.26,67.69 8.26,69.22 6.86,70.61 U$15.1
N$18
  Top 0.305: U$27.14 55.12,30.08 55.12,23.37 58.17,20.32 58.17,14.48 53.34,9.65 U$44.3
N$19
  Top 0.203: R93.2 46.04,37.78 44.99,36.73 U$24.2
N$20
  Top 0.203: R82.2 R4.1
N$21
  Top 0.203: 44.32,35.96 U$24.3 44.34,37.32 44.32,37.34 44.32,39.12 43.81,39.62 R94.2
N$22
  Top 0.203: R83.2 33.88,38.23 R3.1
N$23
  Top 0.305: U$24.11 42.39,28.16 41.66,27.43 34.99,27.43 U$3.P$1
N$24
  Top 0.305: U$24.10 41.74,28.91 41.27,28.45 37.85,28.45 U$4.P$1
N$25
  Top 0.305: U$27.16 56.43,27.26 62.23,21.46 U$42.3
N$26
  Top 0.203: R2.1 50.48,45.25 R15.2
N$27
  Top 0.203: R1.1 52.7,45.38 R16.2
N$28
  Top 0.305: U$27.11 53.18,28.55 52.2,27.56 U$5.P$1
N$29
  Top 0.305: U$27.10 52.53,29.04 52.07,28.57 51.31,28.57 U$10.P$1
N$32
  Top 0.203: R3.2 35.71,38.23 41.15,38.23 42.39,36.99 U$24.6
N$33
  Top 0.203: R4.2 36.83,35.94 38.61,37.72 40.64,37.72 41.74,36.62 U$24.7
N$34
  Top 0.203: R2.2 50.42,41 50.42,39.12 51.44,38.1 51.82,38.1 52.53,37.38 U$27.7
N$35
  Top 0.203: R1.2 52.7,38.1 53.18,37.62 U$27.6
N$44  (via drill 0.3)
  Top 1.016: R26.2 U$13.1 | R25.1 v11.56,80.01 R22.1
  Bottom 1.016: v11.56,80.01 9.14,82.42 9.14,83.31 6.6,85.85 U$13.1
N$58
  Top 0.762: R18.1 5.12,5.12 H1.B3,0
N$59
  Top 0.762: R19.1 11.43,96.52 H3.B3,0
N$60
  Top 0.762: R20.1 94.49,98.55 H4.B3,0
N$61
  Top 0.203: R95.2 39.37,41 39.37,39.75 39.75,39.37 42.42,39.37 43.69,38.1 U$24.4
N$62  (via drill 0.3)
  Top 0.762: R23.2 v39.12,70.48
  Bottom 0.508: U$1.P$1 29.21,67.31 35.94,67.31 v39.12,70.48
N$63
  Top 0.762: R21.1 94.61,9.4 96.52,7.49 H2.B3,0
N$64  (via drill 0.3)
  Top 1.016: R34.2 7.66,55.37 U$16.1 | v13.34,51.18 12.36,51.18 R32.1 R33.1
  Bottom 1.016: v13.34,51.18 10.03,51.18 8.64,52.58 8.64,54.1 7.37,55.37 U$16.1
N$65  (via drill 0.3)
  Top 1.016: R24.2 v30.48,84.96
  Bottom 1.016: v30.48,84.96 U$1.P$11
N$69  (via drill 0.3)
  Top 1.016: R35.1 v11.68,38.1 R36.1 | R37.2 7.58,40.13 U$17.1
  Bottom 1.016: v11.68,38.1 9.65,40.13 U$17.1
N$70  (via drill 0.3)
  Top 1.016: R40.2 5.55,24.89 U$18.1 | v12.95,25.53 11.34,25.53 R38.1 11.3,24.47 R39.1
  Bottom 1.016: v12.95,25.53 12.32,24.89 U$18.1
N$78  (via drill 0.3)
  Top 1.016: U$19.1 96.61,78.07 R43.2 | R42.1 88.65,83.4 88.65,82.8 88.01,82.17 v87.5,82.17 87.67,82.17 R41.1
  Bottom 1.016: v87.5,82.17 91.44,78.23 U$19.1
N$79  (via drill 0.3)
  Top 1.016: U$20.1 92.37,62.99 R46.2 | R45.1 88.14,68.33 v87.38,67.56 87.38,67.48 R44.1
  Bottom 1.016: v87.38,67.56 91.95,62.99 U$20.1
N$80  (via drill 0.3)
  Top 1.016: R51.2 92.8,47.75 U$21.1 | R47.1 86.87,55.16 v86.87,57.4 87.63,58.17 R50.1
  Bottom 1.016: v86.87,57.4 92.96,51.31 92.96,49.4 94.61,47.75 U$21.1
N$81  (via drill 0.3)
  Top 1.016: R54.2 90.46,34.92 91.95,34.92 94.36,32.51 U$22.1 | R52.1 90.83,38.59 | 90.83,38.59 91.1,38.86 v91.82,38.86 | R53.1 90.83,39.14 90.83,38.59
  Bottom 1.016: v91.82,38.86 91.95,38.73 91.95,34.92 94.36,32.51 U$22.1
N$82  (via drill 0.3)
  Top 1.016: R57.2 91.99,17.27 U$23.1 | R55.1 v91.82,26.67 R56.1
  Bottom 1.016: v91.82,26.67 91.82,18.8 93.34,17.27 U$23.1
N$106
  Top 0.203: IC4.12 58.41,84.47 58.1,84.77 56.83,84.77 56.52,85.09 R70.1
N$107
  Top 0.203: IC4.10 59.7,84.44 59.05,85.09 R69.1
N$108
  Top 0.203: IC4.8 61.01,84.5 61.59,85.09 R68.1
N$109
  Top 0.203: IC4.6 60.35,76.81 60.64,76.52 61.28,76.52 61.59,76.2 R67.1
N$110
  Top 0.203: IC4.13 57.76,81.48 57.96,81.28 73.41,81.28 80.26,74.42 84.42,74.42 R125.2 86.21,74.46 C36.1 86.37,74.3 87.25,74.3 87.5,74.55 R132.1
N$111
  Top 0.203: IC4.11 59.05,81.99 59.26,81.79 75.44,81.79 78.49,78.74 84.42,78.74 R124.2 arc45 84.52,78.75 C35.1 86.37,78.74 87.5,78.74 87.76,78.99 R131.1
N$112
  Top 0.203: R75.2 arc-45 84.52,85.2 C32.1 87.47,85.2 arc45 87.61,85.26 87.95,85.6 R130.1 | IC4.9 60.35,82.5 60.56,82.3 81.28,82.3 82.3,83.31 82.3,84.33 83.15,85.18 R75.2 | 84.29,85.34 R75.2
N$113
  Top 0.203: R129.1 88.03,60.2 arc45 87.89,60.14 87.63,59.88 86.52,59.88 arc-45 86.38,59.94 C33.1 84.52,59.96 arc-45 R76.2 84.42,59.94 83.06,59.94 82.3,60.71 82.3,65.53 68.33,79.5 59.91,79.5 59.7,79.3 IC4.5
N$114
  Top 0.203: R96.2 36.32,39.79 36.32,39.75 36.58,39.5 38.61,39.5 39.24,38.86 42.16,38.86 43.04,37.99 U$24.5
N$115
  Top 0.203: IC4.3 58.41,79.81 58.61,80.01 69.09,80.01 82.8,66.29 84.42,66.29 R123.2 arc-45 84.52,66.28 C34.1 86.54,66.28 R128.1
N$116
  Top 0.203: IC4.1 57.1,80.31 57.31,80.52 70.61,80.52 82.3,68.83 84.42,68.83 R126.2 86.33,68.87 C37.1 86.37,68.83 87,68.83 88.52,70.36 R127.1
N$122
  Top 0.305: U$27.15 55.78,26 59.94,21.84 59.94,14.35 64.77,9.53 U$43.3
N$124
  Top 0.305: U$27.13 54.48,24.26 50.8,20.57 U$45.3
N$125
  Top 0.305: U$27.12 53.83,25.26 52.2,23.62 50.29,23.62 47.5,20.83 47.5,14.48 41.91,8.89 U$46.3
N$126
  Top 0.305: U$24.16 45.64,23.79 44.83,22.99 40.77,22.99 39.37,21.59 U$47.3
N$127
  Top 0.305: U$24.15 44.99,26.19 43.18,24.38 39.37,24.38 36.83,21.84 36.83,14.99 30.48,8.64 U$48.3
N$129
  Top 0.305: U$24.13 43.69,26.92 42.67,25.91 37.72,25.91 34.29,22.48 27.81,22.48 25.53,20.19 25.53,14.99 19.05,8.51 U$50.3
N$130
  Top 0.305: U$24.12 43.04,27.42 42.29,26.67 37.08,26.67 34.04,23.62 26.42,23.62 23.62,20.83 17.53,20.83 16.51,19.81 U$51.3
N$131
  Top 0.203: R88.2 63.63,37.34 63.25,36.96 56.01,36.96 55.78,36.73 U$27.2
N$132
  Top 0.203: R89.2 59.37,38.04 58.8,37.47 55.75,37.47 55.13,36.84 U$27.3
N$133
  Top 0.203: R90.2 57.15,38.48 56.64,37.97 55.63,37.97 54.48,36.83 U$27.4
N$134
  Top 0.203: R91.2 54.86,41 54.86,38.48 53.83,37.45 U$27.5
N$163
  Top 0.203: IC6.12 58.41,63.52 57.91,64.01 56.64,64.01 56.39,64.26 56.39,65.06 R138.1
N$164
  Top 0.203: IC6.10 59.7,63.48 59.05,64.14 R137.1
N$165
  Top 0.203: IC6.8 61.01,63.55 61.59,64.14 R136.1
N$167  (via drill 0.3)
  Top 0.203: R150.1 86.25,44.32 arc45 86.11,44.26 85.85,44.01 84.74,44.01 arc-45 84.6,44.06 C43.1 82.74,44.08 arc-45 R143.2 82.59,44.2 80.77,44.2 78.99,45.97 78.99,58.67 v75.44,62.23 | IC6.13 57.76,61.37 59.18,59.94 66.29,59.94 v66.8,60.45
  Bottom 0.203: v66.8,60.45 68.58,62.23 v75.44,62.23
N$168  (via drill 0.3)
  Top 0.203: R149.1 85.85,48.9 85.46,49.29 C42.1 84.56,49.31 R142.2 82.64,49.28 80.77,49.28 79.76,50.29 79.76,60.45 v75.44,64.77 | IC6.11 59.05,61.85 60.45,60.45 65.02,60.45 v65.53,60.96
  Bottom 0.203: v65.53,60.96 65.53,61.21 69.09,64.77 v75.44,64.77
N$169  (via drill 0.3)
  Top 0.203: IC6.9 60.35,61.56 60.96,60.96 64.01,60.96 v64.52,61.47 | R148.1 86.11,53.09 85.85,53.34 84.72,53.34 C39.1 84.56,53.51 R139.2 82.51,53.34 81.28,53.34 80.52,54.1 80.52,62.99 76.2,67.31 v75.44,67.31
  Bottom 0.203: v64.52,61.47 64.52,62.23 69.6,67.31 v75.44,67.31
N$170
  Top 0.203: IC6.5 59.7,57.67 60.2,58.17 62.74,58.17 63.75,57.15 75.18,57.15 76.71,55.63 76.71,35.31 79.46,32.55 R140.2 arc45 82.74,32.53 C40.1 86.13,32.53 R147.1
N$171  (via drill 0.3)
  Top 0.203: IC6.3 58.41,58.15 58.93,58.67 64.01,58.67 64.52,58.17 v68.58,58.17 | v76.96,57.15 77.22,57.15 77.47,56.9 77.47,39.12 80.01,36.58 82.64,36.58 R141.2 84.56,36.62 C41.1 86.13,36.59 R146.1
  Bottom 0.203: v68.58,58.17 69.09,58.17 70.1,57.15 v76.96,57.15
N$172  (via drill 0.3)
  Top 0.203: R145.1 86.17,40.39 85.93,40.15 C44.1 82.7,40.15 R144.2 79.97,40.17 78.23,41.91 78.23,57.4 75.95,59.69 v75.44,59.69 | IC6.1 57.1,58.63 57.66,59.18 v68.58,59.18
  Bottom 0.203: v68.58,59.18 69.6,59.18 70.1,59.69 v75.44,59.69
N$179
  Top 0.203: IC7.12 41.92,76.82 42.23,76.52 43.81,76.52 44.13,76.2 R156.1
N$180
  Top 0.203: IC7.10 40.62,76.85 40.96,76.52 41.27,76.52 41.59,76.2 R155.1
N$181
  Top 0.203: IC7.8 39.33,76.47 39.05,76.2 R154.1
N$182
  Top 0.203: IC7.6 39.98,84.48 39.37,85.09 39.05,85.09 38.73,85.41 R153.1
N$183
  Top 0.203: R168.1 17.06,68.07 R161.2 19.15,68.29 C50.1 20.31,68.31 32.77,80.77 41.91,80.77 42.58,80.11 IC7.13
N$184
  Top 0.203: IC7.11 41.27,79.88 40.89,80.26 33.78,80.26 22.61,69.09 22.61,64.26 20.21,61.86 C49.1 19.21,61.89 R160.2 16.98,61.85 15.75,61.85 15.33,62.27 R167.1
N$185
  Top 0.203: R166.1 14.95,53.87 15.37,54.29 17.17,54.29 R157.2 19.15,54.19 C46.1 19.18,59.31 23.5,63.63 23.5,67.94 35.31,79.76 39.62,79.76 39.98,79.41 IC7.9
N$186
  Top 0.203: R165.1 16,83.06 16.32,83.38 17.17,83.38 R158.2 19.15,83.27 C47.1 36.59,83.3 37.34,82.55 40.39,82.55 40.62,82.79 IC7.5
N$187
  Top 0.203: R164.1 14.95,78.38 15.37,78.8 17.17,78.8 R159.2 19.15,78.7 C48.1 21.58,78.73 24.89,82.04 41.4,82.04 41.92,82.56 IC7.3
N$188
  Top 0.203: R163.1 15.68,73.41 16,73.72 17.17,73.72 R162.2 19.15,73.62 C51.1 23.86,73.65 31.75,81.53 42.67,81.53 43.23,82.09 IC7.1
N$195
  Top 0.203: IC8.12 42.88,55.87 43.18,55.56 44.45,55.56 44.77,55.24 R174.1
N$196
  Top 0.203: IC8.10 41.58,55.9 42.23,55.24 R173.1
N$197
  Top 0.203: IC8.8 40.28,55.84 39.69,55.24 R172.1
N$198
  Top 0.203: IC8.6 40.93,63.53 40.64,63.82 40.32,63.82 39.69,64.45 R171.1
N$199  (via drill 0.3)
  Top 0.203: R186.1 15.88,34.54 16.19,34.86 17.68,34.86 R179.2 19.66,34.76 C57.1 19.7,34.8 21.34,34.8 24.38,37.85 24.38,55.88 v25.65,57.15 | IC8.13 43.53,59.34 43.18,59.69 v36.32,59.69
  Bottom 0.203: v25.65,57.15 33.78,57.15 v36.32,59.69
N$200  (via drill 0.3)
  Top 0.203: R185.1 14.82,30.63 15.24,31.05 17.68,31.05 R178.2 19.66,30.95 C56.1 20.88,30.97 25.15,35.24 v25.15,54.36 | IC8.11 42.23,58.86 41.91,59.18 37.08,59.18 v34.54,56.64
  Bottom 0.203: v34.54,56.64 32.51,54.61 27.18,54.61 26.67,55.12 25.91,55.12 v25.15,54.36
N$201
  Top 0.203: IC8.9 40.93,58.13 40.64,58.42 38.1,58.42 34.29,54.61 26.67,54.61 25.91,53.85 25.91,29.97 22.61,26.67 19.83,26.67 C53.1 19.66,26.5 R175.2 17.57,26.29 16.51,26.29 16.42,26.38 R184.1
N$202  (via drill 0.3)
  Top 0.203: IC8.5 41.58,61.64 41.4,61.47 38.86,61.47 v37.34,62.99 | v24.89,64.26 24.89,63.75 21.08,59.94 21.08,49.64 20.57,49.13 C54.1 19.66,49.11 R176.2 16.6,49.11 16,48.51 R183.1
  Bottom 0.203: v24.89,64.26 25.4,64.77 35.56,64.77 v37.34,62.99
N$203  (via drill 0.3)
  Top 0.203: R182.1 17.57,43.43 R177.2 19.66,43.65 C55.1 19.7,43.69 21.59,43.69 22.35,44.45 22.35,58.93 v25.15,61.72 | IC8.3 42.88,61.42 42.42,60.96 38.1,60.96 v37.34,61.72
  Bottom 0.203: v25.15,61.72 25.65,62.23 34.54,62.23 35.05,61.72 v37.34,61.72
N$204  (via drill 0.3)
  Top 0.203: R181.1 14.82,39.27 15.24,39.69 17.68,39.69 R180.2 17.8,39.61 C58.1 19.7,39.62 22.35,39.62 23.37,40.64 23.37,57.15 v25.4,59.18 | IC8.1 44.18,60.94 43.69,60.45 v37.34,60.45
  Bottom 0.203: v25.4,59.18 25.91,59.69 34.8,59.69 35.56,60.45 v37.34,60.45
SEN_IN0
  Top 0.203: U$18.3 7.62,19.81 10.33,22.52 R39.2 11.6,22.48 12.95,22.48 13.72,23.24 14.61,23.24 15.24,23.88 R184.2
SEN_IN1
  Top 0.203: U$18.2 4.95,22.48 7.75,22.48 9.27,24 9.27,26.29 10.25,27.27 R38.2 11.34,27.3 12.45,27.3 13.12,27.98 R185.2
SEN_IN2
  Top 0.203: R181.2 13.37,35.6 12.83,35.05 11.77,35.05 R36.2 11.6,35.05 U$17.3
SEN_IN3
  Top 0.203: U$17.2 9.4,37.59 10.29,38.48 10.29,40.39 11.01,41.11 R35.2 11.77,41.02 12.7,41.02 13.12,41.44 R182.2
SEN_IN4
  Top 0.203: U$16.3 8,50.29 9.99,48.3 R33.2 13.41,48.3 R183.2
SEN_IN5
  Top 0.203: U$16.2 8.38,52.83 9.23,53.68 R32.2 11.77,53.47 R166.2
SEN_IN6
  Top 0.203: U$15.3 4.95,65.41 8.26,65.41 10.63,63.03 R30.2 13.29,63.03 R167.2
SEN_IN7
  Top 0.203: U$15.2 7.75,68.07 8.09,68.41 R29.2 11.94,70.74 12.61,71.41 R163.2
SEN_IN8
  Top 0.203: U$13.3 7.75,80.77 8.38,80.14 8.38,77.6 9.11,76.87 R25.2 11.6,76.83 12.19,76.83 12.57,77.22 R164.2
SEN_IN9
  Top 0.203: U$13.2 9.14,83.31 9.23,83.4 R22.2 11.6,83.44 12.32,83.44 12.7,83.06 R165.2
SEN_IN10
  Top 0.203: R147.2 87.84,31.54 90.3,29.08 90.3,24.38 90.77,23.91 R55.2 91.95,23.79 91.95,22.35 94.49,19.81 U$23.2
SEN_IN11
  Top 0.203: U$23.3 94.61,22.35 93.47,23.5 93.47,28.96 92.88,29.55 R56.2 90.97,29.55 89.28,31.24 89.28,33.27 87.84,34.71 R146.2
SEN_IN12
  Top 0.203: U$22.2 94.36,35.05 92.92,36.49 R52.2 90.39,36.45 89.53,36.45 89.03,36.96 89.03,38.35 88.61,38.77 R145.2
SEN_IN13
  Top 0.203: U$22.3 93.98,37.59 92.96,38.61 92.96,40.26 91.99,41.24 R53.2 90.42,45.09 88.61,46.9 R149.2
SEN_IN14
  Top 0.203: U$21.2 94.23,50.29 91.44,53.09 R148.2 R47.2
SEN_IN15
  Top 0.203: U$21.3 94.36,52.83 93.47,53.72 93.47,57.4 92.71,58.17 R50.2 R129.2
SEN_IN16
  Top 0.203: U$20.2 93.22,65.53 92.58,66.17 R44.2 R128.2
SEN_IN17
  Top 0.203: R127.2 R45.2 91.69,68.33 91.95,68.07 U$20.3
SEN_IN18
  Top 0.203: U$19.2 96.65,80.64 93.09,80.64 92.58,81.15 R41.2 R131.2
SEN_IN19
  Top 0.203: U$19.3 93.6,83.31 93.47,83.44 R42.2 R130.2
SOL0_EN
  Top 0.203: R92.1 48.26,43.94 48.77,44.45 48.77,45.31 R122.2 47.78,45.44 47.24,45.97 47.24,48.77 46.74,49.28 33.78,49.28 32.26,50.8 U$1.P$18
SOL0_INA
  Top 0.203: R169.2 44.77,68.52 44.45,68.83 37.08,68.83 35.31,67.06 35.31,62.23 31.5,58.42 U$1.P$15
SOL0_INB
  Top 0.203: R170.2 42.23,68.01 41.91,68.33 37.59,68.33 35.81,66.55 35.81,61.47 31.5,57.15 29.21,57.15 U$1.P$6
SOL1_EN
  Top 0.203: U$1.P$8 29.21,49.53 32.77,49.53 33.78,48.51 44.2,48.51 44.7,48.01 44.7,45.97 45.21,45.47 45.87,45.47 R121.2 45.97,45.44 45.97,44.2 46.04,44.13 R93.1
SOL1_INA
  Top 0.203: R171.2 37.49,67.21 36.32,66.04 36.32,60.96 33.78,58.42 33.78,57.66 32,55.88 U$1.P$16
SOL1_INB
  Top 0.203: R172.2 36.09,52.81 35.56,53.34 U$1.P$17
SOL2_EN
  Top 0.203: R94.1 42.84,42.76 42.67,42.93 42.67,43.18 42.42,43.43 41.55,43.43 R86.2 41.53,47.12 40.89,47.75 32.26,47.75 31.75,48.26 U$1.P$19
SOL2_INA
  Top 0.203: R173.2 42.23,50.35 41.91,50.04 35.31,50.04 33.27,52.07 29.21,52.07 U$1.P$7
SOL2_INB  (via drill 0.3)
  Top 0.203: R151.2 44.45,89.15 43.94,89.66 35.56,89.66 34.29,88.39 v34.29,85.34 | U$1.P$2 29.21,67.31 29.21,69.34 34.29,74.42 v34.29,76.96
  Bottom 0.203: v34.29,85.34 v34.29,76.96
SOL3_EN
  Top 0.203: U$1.P$9 27.94,47.75 28.7,46.99 36.07,46.99 37.21,45.85 R85.2 38.08,43.46 38.35,43.18 38.35,42.93 38.61,42.67 39.22,42.67 R95.1
SOL3_INA  (via drill 0.3)
  Top 0.203: U$1.P$3 29.21,64.77 31.5,64.77 32.26,65.53 32.26,70.61 35.31,73.66 v35.31,77.72 | R152.2 41.59,88.71 41.15,89.15 36.32,89.15 35.31,88.14 v35.31,84.33
  Bottom 0.203: v35.31,84.33 v35.31,77.72
SOL3_INB  (via drill 0.3)
  Top 0.203: 37.08,87.88 38.7,87.88 R153.2 37.05,87.84 36.32,87.12 v36.32,85.34 | v36.32,78.74 36.32,73.15 33.02,69.85 33.02,64.77 31.75,63.5 U$1.P$13
  Bottom 0.203: v36.32,85.34 v36.32,78.74
SOL4_EN
  Top 0.203: R96.1 34.99,42.7 R84.2 32.87,42.67 28.7,42.67 27.94,43.43 U$1.P$10
SOL4_INA
  Top 0.203: R154.2 39.01,73.41 37.85,73.41 33.78,69.34 33.78,63.5 31.24,60.96 U$1.P$14
SOL4_INB
  Top 0.203: R155.2 41.59,72.33 41.15,71.88 38.35,71.88 34.54,68.07 34.54,62.99 31.24,59.69 29.21,59.69 U$1.P$5
SOL5_EN
  Top 0.203: R87.1 67.94,42.7 R77.2 72.54,42.7 73.66,43.81 U$1.P$40
SOL5_INA
  Top 0.203: R133.2 56.52,51.31 57.4,50.42 65.02,50.42 67.94,53.34 U$1.P$27
SOL5_INB
  Top 0.203: R134.2 59.05,51.44 59.44,51.05 64.52,51.05 65.72,52.26 66.04,52.58 68.07,54.61 72.39,54.61 U$1.P$36
SOL6_EN
  Top 0.203: R88.1 63.69,42.7 R81.2 65.79,43.56 66.17,43.94 71.37,43.94 72.39,44.96 72.39,46.99 U$1.P$39
SOL6_INA
  Top 0.203: R135.2 63.67,52.49 64.01,52.83 64.01,55.12 64.77,55.88 U$1.P$26
SOL6_INB
  Top 0.203: U$1.P$25 62.65,66.89 R136.2
SOL7_EN
  Top 0.203: R89.1 61.4,42.76 R80.2 63.35,44.58 67.94,44.58 68.71,45.34 68.71,48.01 70.23,49.53 72.39,49.53 U$1.P$38
SOL7_INA
  Top 0.203: R137.2 59.05,67.82 59.44,68.2 62.61,68.2 69.85,60.96 U$1.P$24
SOL7_INB
  Top 0.203: R65.2 56.52,69.22 56.9,68.83 63.5,68.83 70.1,62.23 72.39,62.23 U$1.P$33
SOL8_EN
  Top 0.203: R90.1 57.15,44.2 58.29,45.34 66.04,45.34 67.06,46.35 67.06,47.85 R79.2 70,50.8 U$1.P$28
SOL8_INA
  Top 0.203: R66.2 59.05,70.74 60.2,69.6 63.37,69.6 64.26,69.6 65.02,69.6 U$1.P$23
SOL8_INB
  Top 0.203: R67.2 61.59,71.25 62.48,70.36 66.55,70.36 69.72,67.18 72.52,67.18 U$1.P$32
SOL9_EN
  Top 0.203: R91.1 54.93,45.72 56.96,47.75 R78.2 61.06,49 61.47,49.4 66.8,49.4 69.47,52.07 72.39,52.07 U$1.P$37
SOL9_INA  (via drill 0.3)
  Top 0.203: R68.2 63.03,87.84 63.25,87.63 v63.25,83.31 | v63.25,78.74 63.25,76.71 66.29,73.66 68.58,73.66 71.12,71.12 U$1.P$21
  Bottom 0.203: v63.25,83.31 v63.25,78.74
SOL9_INB  (via drill 0.3)
  Top 0.203: R69.2 59.05,89.03 57.91,90.17 35.05,90.17 33.53,88.65 v33.53,84.33 | v33.02,76.2 33.02,75.44 26.42,68.83 26.42,62.48 U$1.P$4
  Bottom 0.203: v33.53,84.33 33.53,77.72 33.02,77.22 v33.02,76.2

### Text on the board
Bottom: 900101 rev A
tPlace: 900100 REV | GND | +5V | +3.3V | IN8 | IN9 | IN6 | IN7 | IN4 | IN5 | IN2 | IN3 | IN0 | IN1 | OUT1 | OUT3 | OUT5 | OUT7 | OUT9 | OUT0 | OUT2 | OUT4 | OUT6 | OUT8 | 24VDC | + | - | 24VDC
_tsilk: 900100 | rev | +5V | +3.3V | IN 4 | IN 9 | IN 3 | IN 8 | IN 2 | IN 7 | IN 1 | IN 6 | IN 0 | IN 5 | OUT 4 | OUT 2 | OUT 0 | OUT 8 | OUT 5 | OUT 3 | OUT 1 | OUT 9 | OUT 7 | OUT 6 | +24V DC | +24V | + | -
